(* Logix 5000 AddOnInstructionDefinition export Banner_Q5X_5000_Param_v4; software revision 33.00 *)

TYPE Banner_IOL_Port_v4 :   // UDT that has all of the data items necessary to communicate with a specific Port on a IO-Link Master
STRUCT
   Port_Controlled : INT;   // Each bit represents a port on an IO-Link Master. Set to 1 to tell AOI to control that port.
   Port_Activate : INT;   // Each bit represents a port on an IO-Link Master. When ON that port will process any commands in queue.
   Port_Read : INT;   // Each bit represents a port on an IO-Link Master. Used to determine when device AOI has requested a Read command.
   Port_Write : INT;   // Each bit represents a port on an IO-Link Master. Used to determine when device AOI has requested a Write command.
   Port_RW_Complete : INT;   // Each bit represents a port on an IO-Link Master. Tells device AOI that Read or Write request has been completed.
   Port_Device_Read : INT;
   Data_Transfer : SINT[190];   // Array to transfer data from IO-Master to device AOIs.
END_STRUCT
END_TYPE

TYPE Banner_Q5X_5000_RD_v4 :   // UDT that stores the Write Data for a Q5X 5000.
STRUCT
   Master_Cycle_Time : INT;
   Min_Cycle_Time : INT;
   M_Sequence_Capability : INT;
   IO_Link_Version_ID : INT;
   Process_Data_Input_Length : INT;
   Process_Data_Output_Length : INT;
   Combined_Vendor_ID : DINT;   // IO-Link Vendor ID
   Vendor_ID1 : INT;
   Vendor_ID2 : INT;
   Combined_Device_ID : DINT;   // IO-Link Device ID
   Device_ID1 : INT;
   Device_ID2 : INT;
   Device_ID3 : INT;
   Serial_Number : STRING;
   Teach_State : SINT;
   SP1_TP1 : SINT;
   SP1_TP2 : SINT;
   Measurement_1 : DINT;
   Excess_Gain : DINT;   // Amount of singla measured over the minimum threshold.
   Stability : SINT;
   Emitter_Status : SINT;   // 0 = Active, 1 = Inactive
   Laser_Fault_Status : SINT;   // 0 = No Fault, 1 = Fault Present
   BDC1_Totalizer_Counts : DINT;
   BDC2_Totalizer_Counts : DINT;
   Temperature : DINT;
   Last_Taught_Temperature : DINT;   // Internal Temperature the last time device was taught.
   All_Time_Run_Time : DINT;   // Read only counter that tracks the total time sensor has been running since manufacture. Value in Hours.
   Display : STRING;   // Last Display information
   MDC_Lower_Limit : DINT;
   MDC_Upper_Limit : DINT;
   MDC_Unit : INT;
   MDC_Scale : SINT;
END_STRUCT
END_TYPE

TYPE Banner_Q5X_5000_v4 :   // All of the parameters for a Q5X 5000.
STRUCT
   Initial_Global_Read : BOOL;   // Determines if all of the IO-Link data has been read into the PLC yet
   Command : INT;   // Value placed in here will activate a read or write to a specifc IO-Link Index
   Read : Banner_Q5X_5000_RD_v4;   // Read Only Data
   Write : Banner_Q5X_5000_WD_v4;   // Write Data
   Archive : Banner_Q5X_5000_WD_v4;   // Archive Data
   Reset : BOOL;   // Resets AOI. This will force a complete parameter read of the sensor.
END_STRUCT
END_TYPE

TYPE Banner_Q5X_5000_WD_v4 :   // UDT that stores the Write Data for a Q5X 5000.
STRUCT
   System_Command : INT;   // See IODD file for list of commands that can be activated via the System Command interface
   Parameter_Access_Lock : SINT;   // Write access to all parameters is prohibited while value is 1. Only this parameter can be adjusted when value is 1.
   Data_Storage_Lock : SINT;   // Automatic data storage is disabled when this value is equal to 1. Read access is not affected.
   Local_Parameterization_Lock : SINT;   // Parameterization via local control elements on device is disabled.
   Local_User_Interface_Lock : SINT;   // Operation of local user interface is disabled.
   Teach_in_Channel : SINT;   // 0 = Default, 1 = BDC1, 2 = BDC2
   BDC1_Setpoint_1 : DINT;
   BDC1_Setpoint_2 : DINT;   // In FGS, defines the second switching point. Other modes do not use this parameter.
   BDC1_Switchpoint_Logic : INT;   // 0 = Light Operate, 1 = Dark Operate
   BDC1_Mode : INT;   // 1 = 1Pt BGS, 128 = 2Pt Static BGS, 129 = Dynamic BGS, 130 = 1Pt Window (FGS), 131 = Dual Teach
   BDC1_Hysteresis : INT;   // Hysteresis value for the switchpoint. A value of 0 will result in automatically calculated hysteresis
   BDC2_Setpoint_1 : DINT;
   BDC2_Setpoint_2 : DINT;   // In FGS, defines the second switching point. Other modes do not use this parameter.
   BDC2_Switchpoint_Logic : INT;   // 0 = Light Operate, 1 = Dark Operate
   BDC2_Mode : INT;   // BDC1_Mode SINT Decimal 1 = 1Pt BGS, 128 = 2Pt Static BGS, 129 = Dynamic BGS, 130 = 1Pt Window (FGS), 131 = Dual Teach
   BDC2_Hysteresis : INT;   // Hysteresis value for the switchpoint. A value of 0 will result in automatically calculated hysteresis
   Response_Speed : SINT;   // 0 = Speed 0, 1 = Speed 1, 2 = Speed 2, 3 = Speed 3
   Gain : SINT;   // 0 = Normal, 1 = Best Accuracy, 2 = High Excess Gain
   Secondary_Output_Mode : SINT;   // 0 = Independent Output, 1 = Complementary Output, 2 = Pulse Frequency Output
   Zero_Reference_Location : SINT;   // 0 = Near, 1 = Far
   Shift_Zero_after_Teach : SINT;   // 0 = Off, 1 = On
   Display_Read : SINT;   // 0 = On, 1 = On Inverted, 2 = Off, 3 = Off Inverted
   Display_Units : SINT;   // 0 = Centimeters, 1 = Inches, 2 = Millimeters
   Pushbutton_Lockout : SINT;   // 0 = No Lockout, 1 = Pushbuttons Locked, 2 = Operator Lockout
   Output_Polarity : SINT;   // 0 = Default, 1 = PNP, 2 = NPN
   IOL_Filter_Time : INT;   // Time to average IOl process data measurement between updates
   Include_Binary : SINT;   // 0 = Include, 1 = Don't Include, 2= Measurement Device
   Measurement_1 : SINT;   // 0 = Disabled, 1 = Excess Gain, 2 = Excess Gain / 10, 3 = Channel 1 Dual Mode Percent
   Measurement_2 : SINT;   // 0 = Disabled, 1 = Distance Value, 2 = Displayed Distance, 3 = Channel 2 Dual Mode Percent
   BDC1_Delay_Mode : SINT;   // 0 = Disabled, 1 = On Off Delay, 2 = Oneshot, 3 = Totalizer
   BDC1_Delay_Timer_1 : DINT;   // 0 to 90000
   BDC1_Delay_Timer_2 : DINT;   // 0 to 90000
   BDC1_BGS_Teach_Offset : SINT;   // 0 = Auto, 1 = User Selected
   BDC1_FGS_Window_Size : SINT;   // 0 = Auto, 1 = User Selected
   BDC1_User_Teach_Offset : DINT;   // Mode must be FGS of BGS. Set the user defined offset. Can be positive or negative.
   BDC1_User_FGS_Window_Size : DINT;   // Mode must be FGS. Set the +/- window value.
   BDC1_Auto_Thresholding : SINT;   // 0 = On, 1 = Off, 2 = High Speed
   BDC2_Delay_Mode : SINT;   // 0 = Disabled, 1 = On Off Delay, 2 = Oneshot, 3 = Totalizer
   BDC2_Delay_Timer_1 : DINT;   // 0 to 90000
   BDC2_Delay_Timer_2 : DINT;   // 0 to 90000
   BDC2_BGS_Teach_Offset : SINT;   // 0 = Auto, 1 = User Selected
   BDC2_FGS_Window_Size : SINT;   // 0 = Auto, 1 = User Selected
   BDC2_User_Teach_Offset : DINT;   // Mode must be FGS of BGS. Set the user defined offset. Can be positive or negative.
   BDC2_User_FGS_Window_Size : DINT;   // Mode must be FGS. Set the +/- window value.
   BDC2_Auto_Thresholding : SINT;   // 0 = On, 1 = Off, 2 = High Speed
   Resettable_Run_Time : DINT;
   PFM_Near : DINT;   // 100 to 45000 in Hz
   PFM_Far : DINT;   // 100 to 45000 in Hz
   All_Time_Run_Time_Event_Time : DINT;
   Resettable_Run_Time_Event_Time : DINT;
END_STRUCT
END_TYPE

ADD_ON_INSTRUCTION Banner_Q5X_5000_Param_v4   (* revision 4.1, vendor Banner Engineering *)
// AOI to read and write parameter data to an IO-Link Q5X.
VAR_IN_OUT
   Q5X : Banner_Q5X_5000_v4; {required}
   Port_Data : Banner_IOL_Port_v4; {required}
END_VAR
VAR_INPUT
   Port : DINT; {required}
END_VAR
VAR
   Local_Control : DINT; {access None}
   Global_Read_Command_Value : INT; {access None}
   Global_Write_Command_Value : INT; {access None}
   Command_Being_Processed : BOOL; {access None}
   Update_Archive : BOOL; {access None}
   Index_Write_Inprocess : INT; {access None}
   Index_Write_Control : INT; {access None}
   Inprocess_Index : DINT; {access None}
END_VAR

ROUTINE Logic   (* ladder *)
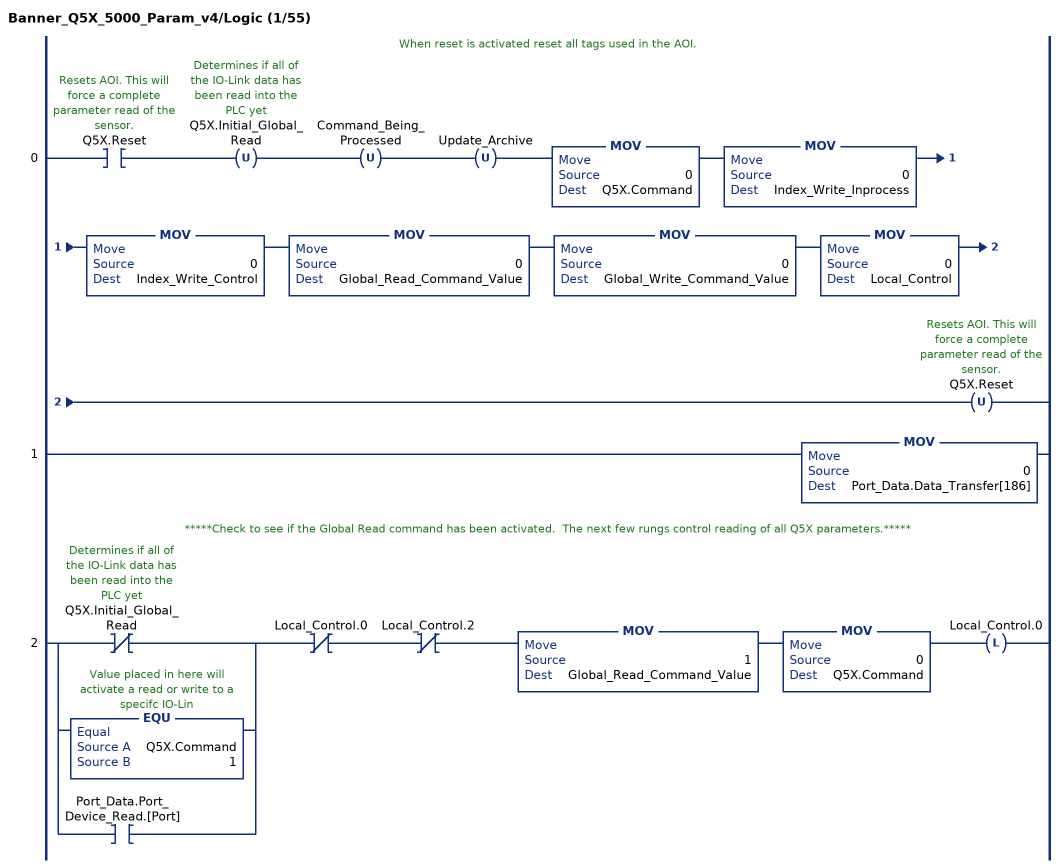
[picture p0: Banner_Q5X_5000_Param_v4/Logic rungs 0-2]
   // When reset is activated reset all tags used in the AOI.
   0: XIC(Q5X.Reset)OTU(Q5X.Initial_Global_Read)OTU(Command_Being_Processed)OTU(Update_Archive)MOV(0,Q5X.Command)MOV(0,Index_Write_Inprocess)MOV(0,Index_Write_Control)MOV(0,Global_Read_Command_Value)MOV(0,Global_Write_Command_Value)MOV(0,Local_Control)OTU(Q5X.Reset);
   1: MOV(0,Port_Data.Data_Transfer[186]);
   // *****Check to see if the Global Read command has been activated.  The next few rungs control reading of all Q5X parameters.*****
   2: [XIO(Q5X.Initial_Global_Read) ,EQU(Q5X.Command,1) ,XIC(Port_Data.Port_Device_Read.[Port]) ]XIO(Local_Control.0)XIO(Local_Control.2)MOV(1,Global_Read_Command_Value)MOV(0,Q5X.Command)OTL(Local_Control.0);
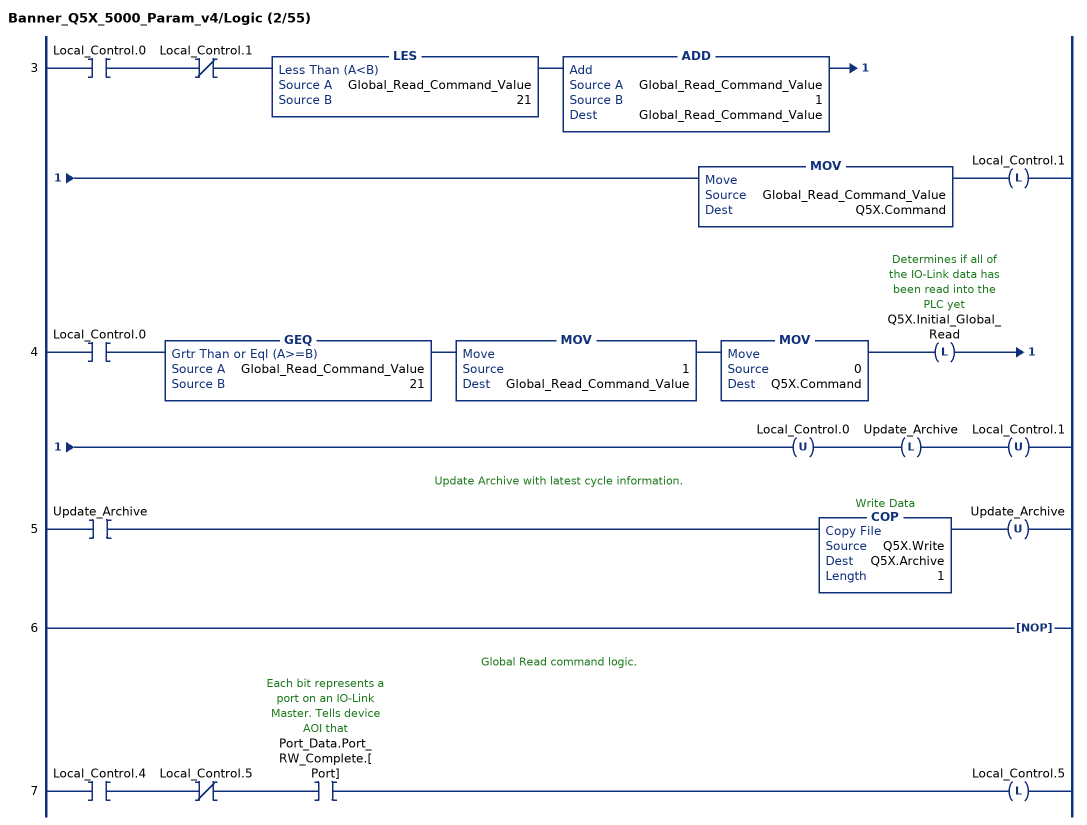
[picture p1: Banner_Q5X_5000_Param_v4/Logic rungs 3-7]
   3: XIC(Local_Control.0)XIO(Local_Control.1)LES(Global_Read_Command_Value,21)ADD(Global_Read_Command_Value,1,Global_Read_Command_Value)MOV(Global_Read_Command_Value,Q5X.Command)OTL(Local_Control.1);
   4: XIC(Local_Control.0)GEQ(Global_Read_Command_Value,21)MOV(1,Global_Read_Command_Value)MOV(0,Q5X.Command)OTL(Q5X.Initial_Global_Read)OTU(Local_Control.0)OTL(Update_Archive)OTU(Local_Control.1);
   // Update Archive with latest cycle information.
   5: XIC(Update_Archive)COP(Q5X.Write,Q5X.Archive,1)OTU(Update_Archive);
   6: NOP();
   // Global Read command logic.
   7: XIC(Local_Control.4)XIO(Local_Control.5)XIC(Port_Data.Port_RW_Complete.[Port])OTL(Local_Control.5);
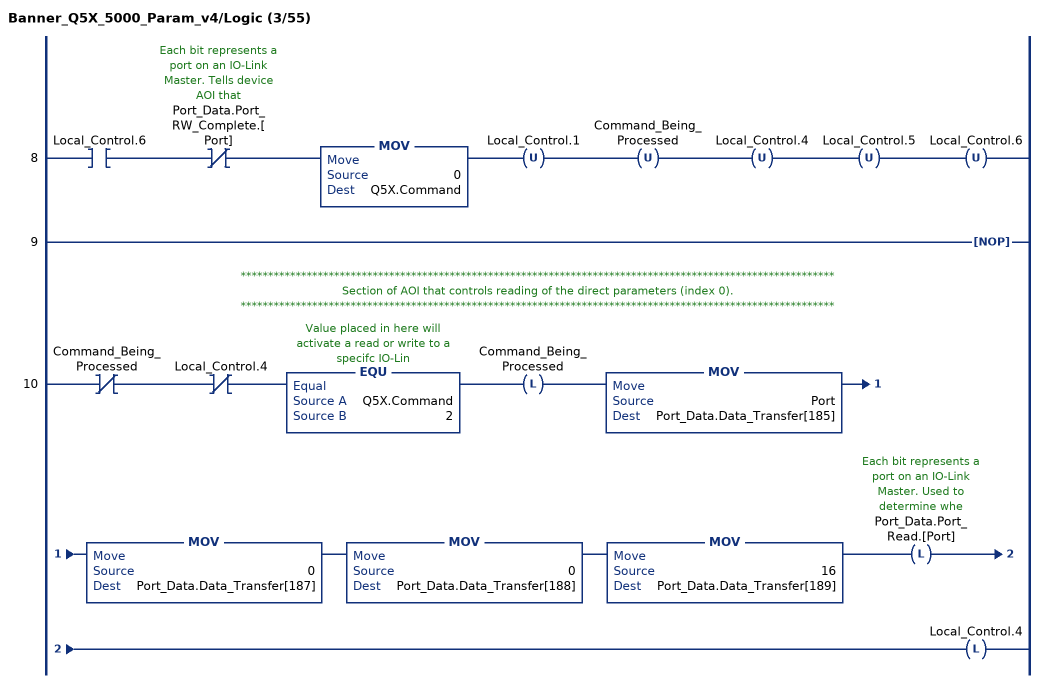
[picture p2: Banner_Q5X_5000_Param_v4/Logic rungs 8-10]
   8: XIC(Local_Control.6)XIO(Port_Data.Port_RW_Complete.[Port])MOV(0,Q5X.Command)OTU(Local_Control.1)OTU(Command_Being_Processed)OTU(Local_Control.4)OTU(Local_Control.5)OTU(Local_Control.6);
   9: NOP();
   // ************************************************************************************************************
   // Section of AOI that controls reading of the direct parameters (index 0).
   // ************************************************************************************************************
   10: XIO(Command_Being_Processed)XIO(Local_Control.4)EQU(Q5X.Command,2)OTL(Command_Being_Processed)MOV(Port,Port_Data.Data_Transfer[185])MOV(0,Port_Data.Data_Transfer[187])MOV(0,Port_Data.Data_Transfer[188])MOV(16,Port_Data.Data_Transfer[189])OTL(Port_Data.Port_Read.[Port])OTL(Local_Control.4);
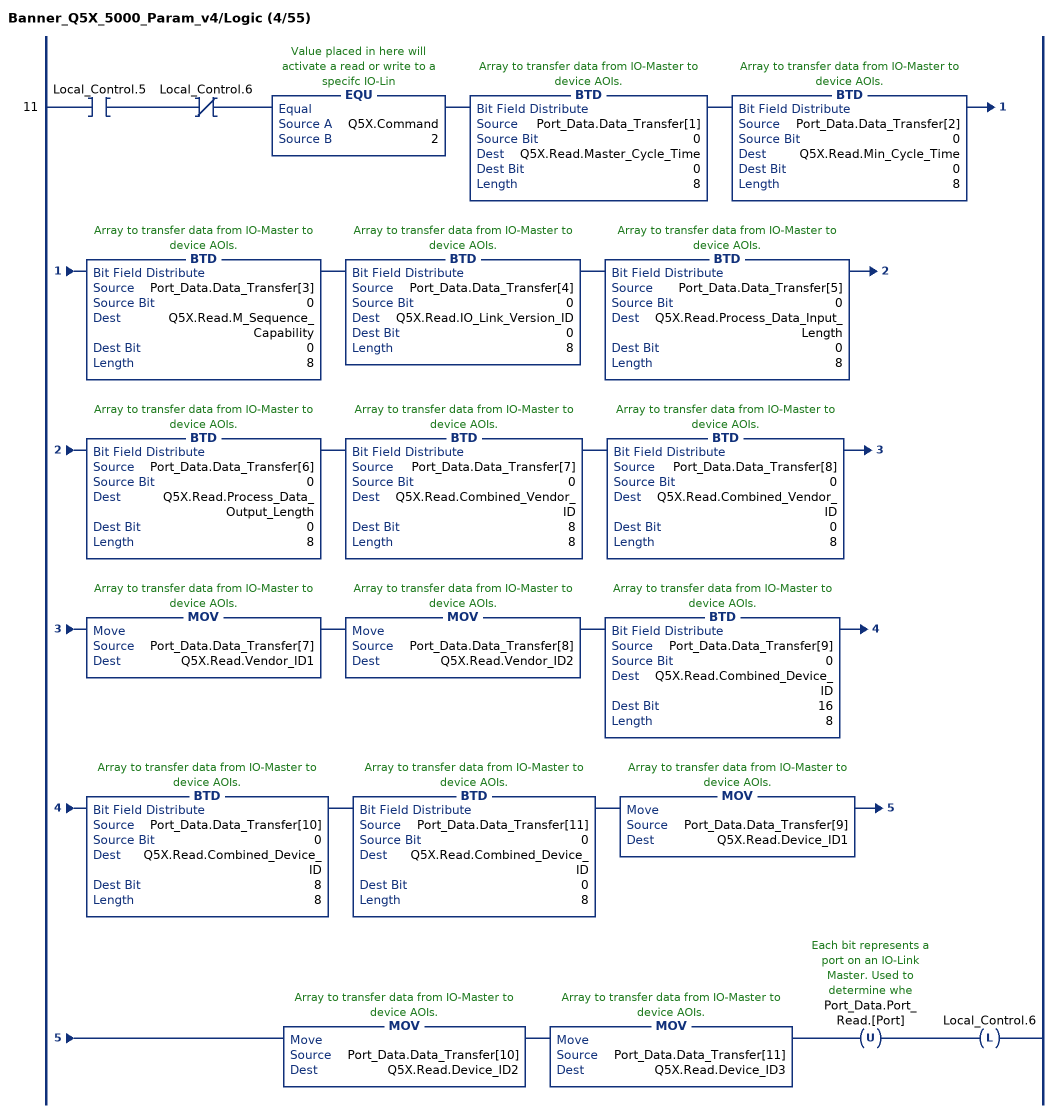
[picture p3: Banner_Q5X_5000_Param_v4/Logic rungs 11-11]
   11: XIC(Local_Control.5)XIO(Local_Control.6)EQU(Q5X.Command,2)BTD(Port_Data.Data_Transfer[1],0,Q5X.Read.Master_Cycle_Time,0,8)BTD(Port_Data.Data_Transfer[2],0,Q5X.Read.Min_Cycle_Time,0,8)BTD(Port_Data.Data_Transfer[3],0,Q5X.Read.M_Sequence_Capability,0,8)BTD(Port_Data.Data_Transfer[4],0,Q5X.Read.IO_Link_Version_ID,0,8)BTD(Port_Data.Data_Transfer[5],0,Q5X.Read.Process_Data_Input_Length,0,8)BTD(Port_Data.Data_Transfer[6],0,Q5X.Read.Process_Data_Output_Length,0,8)BTD(Port_Data.Data_Transfer[7],0,Q5X.Read.Combined_Vendor_ID,8,8)BTD(Port_Data.Data_Transfer[8],0,Q5X.Read.Combined_Vendor_ID,0,8)MOV(Port_Data.Data_Transfer[7],Q5X.Read.Vendor_ID1)MOV(Port_Data.Data_Transfer[8],Q5X.Read.Vendor_ID2)BTD(Port_Data.Data_Transfer[9],0,Q5X.Read.Combined_Device_ID,16,8)BTD(Port_Data.Data_Transfer[10],0,Q5X.Read.Combined_Device_ID,8,8)BTD(Port_Data.Data_Transfer[11],0,Q5X.Read.Combined_Device_ID,0,8)MOV(Port_Data.Data_Transfer[9],Q5X.Read.Device_ID1)MOV(Port_Data.Data_Transfer[10],Q5X.Read.Device_ID2)MOV(Port_Data.Data_Transfer[11],Q5X.Read.Device_ID3)OTU(Port_Data.Port_Read.[Port])OTL(Local_Control.6);
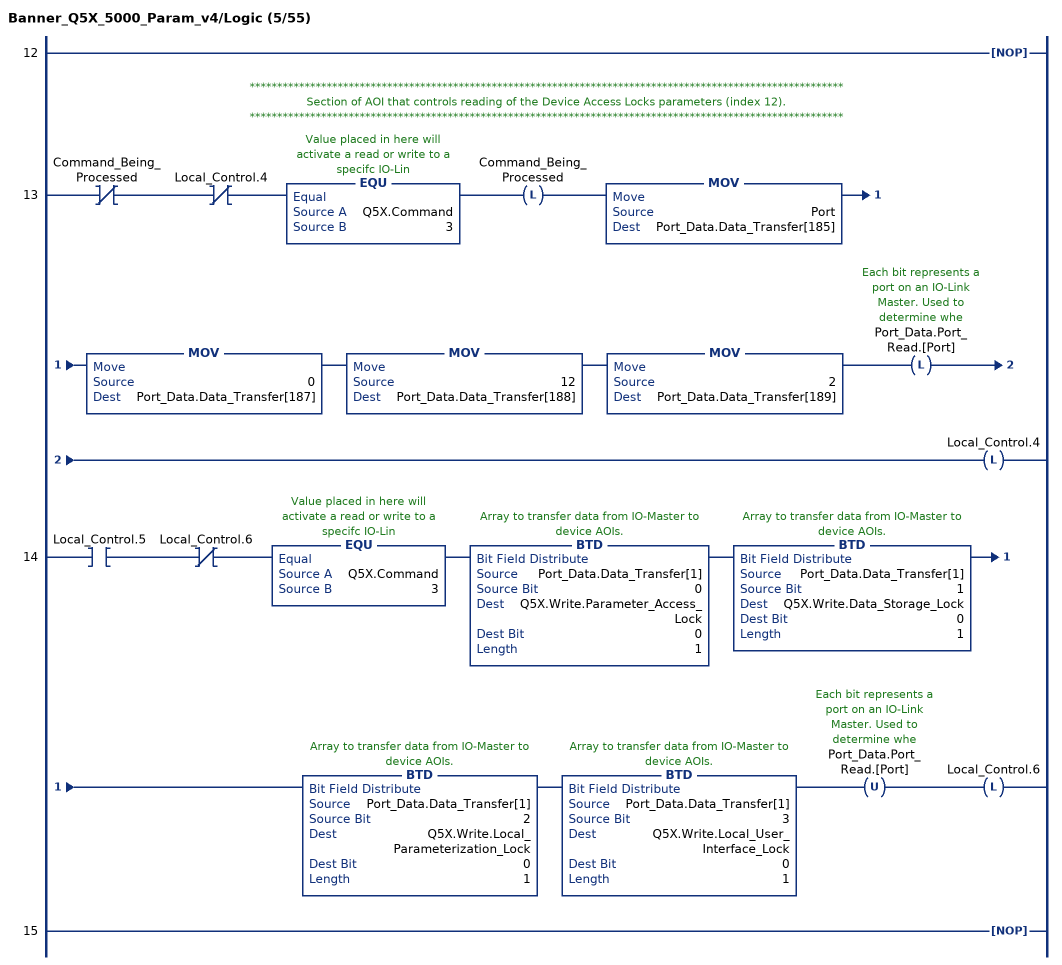
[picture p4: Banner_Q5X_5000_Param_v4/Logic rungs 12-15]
   12: NOP();
   // ************************************************************************************************************
   // Section of AOI that controls reading of the Device Access Locks parameters (index 12).
   // ************************************************************************************************************
   13: XIO(Command_Being_Processed)XIO(Local_Control.4)EQU(Q5X.Command,3)OTL(Command_Being_Processed)MOV(Port,Port_Data.Data_Transfer[185])MOV(0,Port_Data.Data_Transfer[187])MOV(12,Port_Data.Data_Transfer[188])MOV(2,Port_Data.Data_Transfer[189])OTL(Port_Data.Port_Read.[Port])OTL(Local_Control.4);
   14: XIC(Local_Control.5)XIO(Local_Control.6)EQU(Q5X.Command,3)BTD(Port_Data.Data_Transfer[1],0,Q5X.Write.Parameter_Access_Lock,0,1)BTD(Port_Data.Data_Transfer[1],1,Q5X.Write.Data_Storage_Lock,0,1)BTD(Port_Data.Data_Transfer[1],2,Q5X.Write.Local_Parameterization_Lock,0,1)BTD(Port_Data.Data_Transfer[1],3,Q5X.Write.Local_User_Interface_Lock,0,1)OTU(Port_Data.Port_Read.[Port])OTL(Local_Control.6);
   15: NOP();
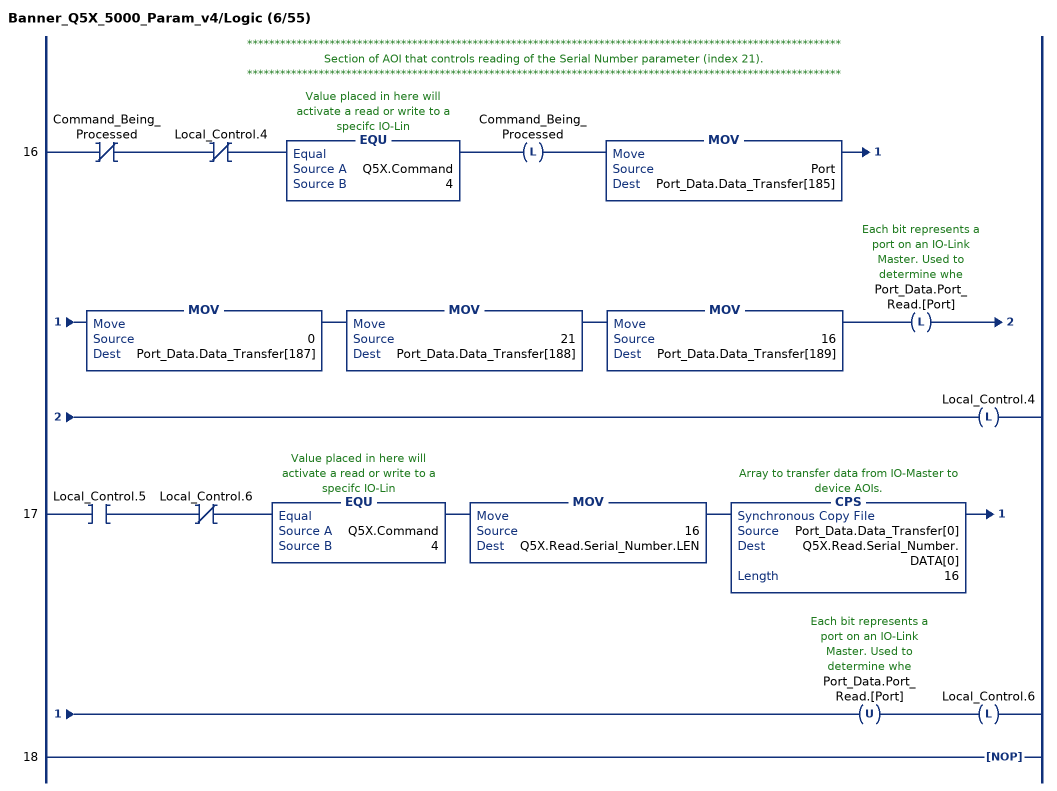
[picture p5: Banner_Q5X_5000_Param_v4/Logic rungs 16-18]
   // ************************************************************************************************************
   // Section of AOI that controls reading of the Serial Number parameter (index 21).
   // ************************************************************************************************************
   16: XIO(Command_Being_Processed)XIO(Local_Control.4)EQU(Q5X.Command,4)OTL(Command_Being_Processed)MOV(Port,Port_Data.Data_Transfer[185])MOV(0,Port_Data.Data_Transfer[187])MOV(21,Port_Data.Data_Transfer[188])MOV(16,Port_Data.Data_Transfer[189])OTL(Port_Data.Port_Read.[Port])OTL(Local_Control.4);
   17: XIC(Local_Control.5)XIO(Local_Control.6)EQU(Q5X.Command,4)MOV(16,Q5X.Read.Serial_Number.LEN)CPS(Port_Data.Data_Transfer[0],Q5X.Read.Serial_Number.DATA[0],16)OTU(Port_Data.Port_Read.[Port])OTL(Local_Control.6);
   18: NOP();
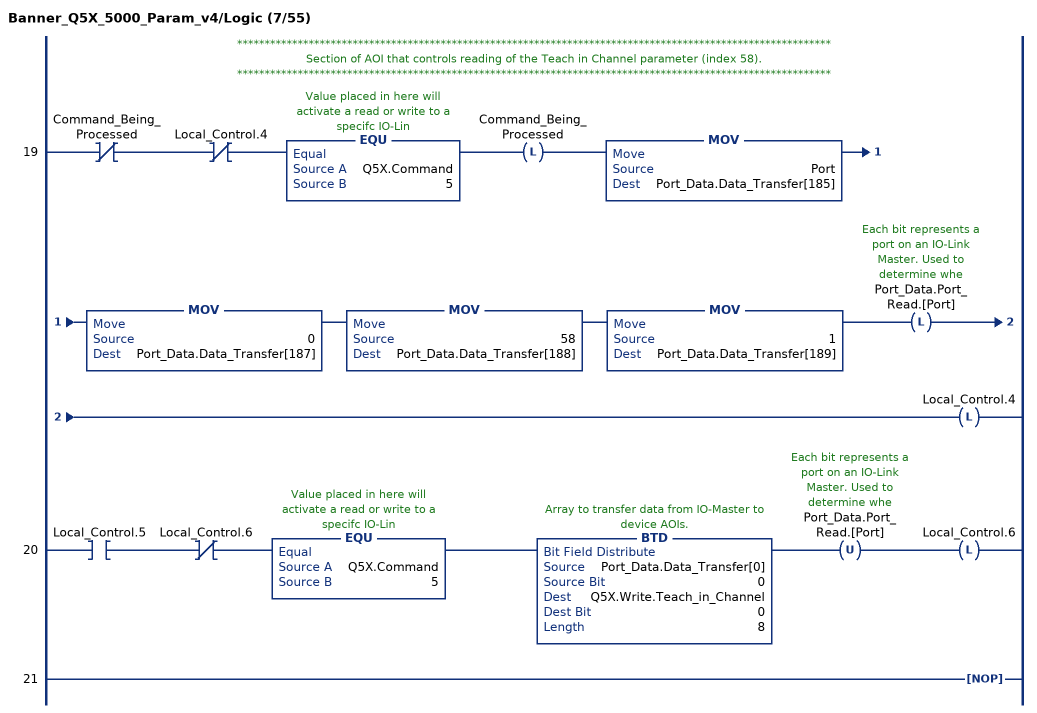
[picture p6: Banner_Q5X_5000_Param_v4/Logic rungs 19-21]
   // ************************************************************************************************************
   // Section of AOI that controls reading of the Teach in Channel parameter (index 58).
   // ************************************************************************************************************
   19: XIO(Command_Being_Processed)XIO(Local_Control.4)EQU(Q5X.Command,5)OTL(Command_Being_Processed)MOV(Port,Port_Data.Data_Transfer[185])MOV(0,Port_Data.Data_Transfer[187])MOV(58,Port_Data.Data_Transfer[188])MOV(1,Port_Data.Data_Transfer[189])OTL(Port_Data.Port_Read.[Port])OTL(Local_Control.4);
   20: XIC(Local_Control.5)XIO(Local_Control.6)EQU(Q5X.Command,5)BTD(Port_Data.Data_Transfer[0],0,Q5X.Write.Teach_in_Channel,0,8)OTU(Port_Data.Port_Read.[Port])OTL(Local_Control.6);
   21: NOP();
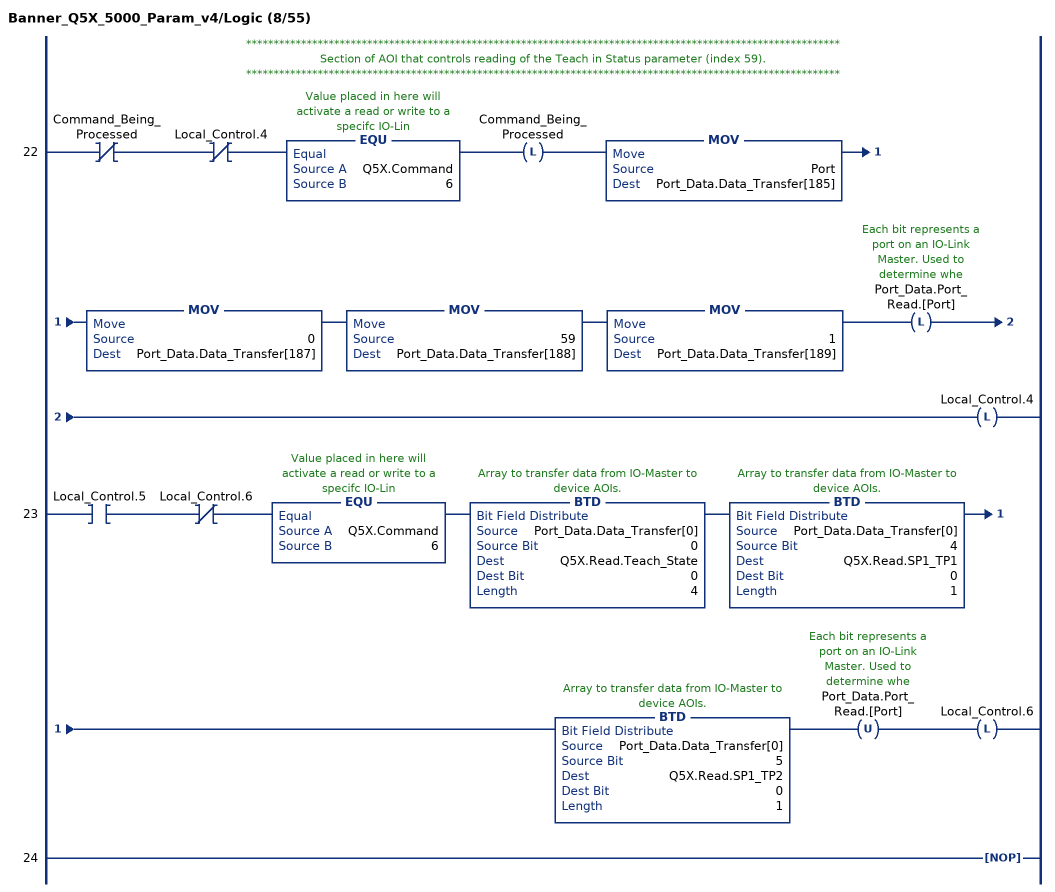
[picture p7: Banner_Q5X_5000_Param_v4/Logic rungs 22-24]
   // ************************************************************************************************************
   // Section of AOI that controls reading of the Teach in Status parameter (index 59).
   // ************************************************************************************************************
   22: XIO(Command_Being_Processed)XIO(Local_Control.4)EQU(Q5X.Command,6)OTL(Command_Being_Processed)MOV(Port,Port_Data.Data_Transfer[185])MOV(0,Port_Data.Data_Transfer[187])MOV(59,Port_Data.Data_Transfer[188])MOV(1,Port_Data.Data_Transfer[189])OTL(Port_Data.Port_Read.[Port])OTL(Local_Control.4);
   23: XIC(Local_Control.5)XIO(Local_Control.6)EQU(Q5X.Command,6)BTD(Port_Data.Data_Transfer[0],0,Q5X.Read.Teach_State,0,4)BTD(Port_Data.Data_Transfer[0],4,Q5X.Read.SP1_TP1,0,1)BTD(Port_Data.Data_Transfer[0],5,Q5X.Read.SP1_TP2,0,1)OTU(Port_Data.Port_Read.[Port])OTL(Local_Control.6);
   24: NOP();
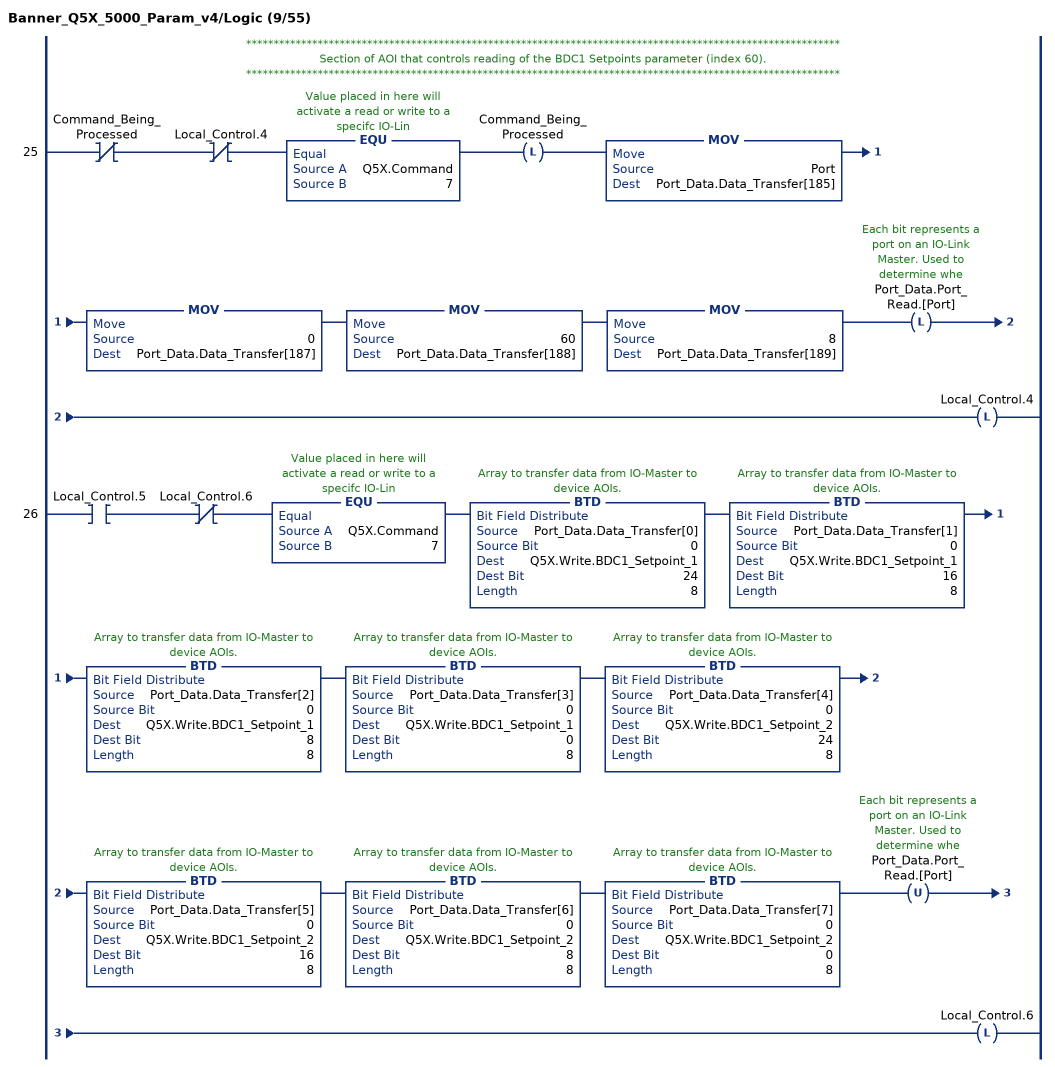
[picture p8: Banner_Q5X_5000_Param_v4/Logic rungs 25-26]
   // ************************************************************************************************************
   // Section of AOI that controls reading of the BDC1 Setpoints parameter (index 60).
   // ************************************************************************************************************
   25: XIO(Command_Being_Processed)XIO(Local_Control.4)EQU(Q5X.Command,7)OTL(Command_Being_Processed)MOV(Port,Port_Data.Data_Transfer[185])MOV(0,Port_Data.Data_Transfer[187])MOV(60,Port_Data.Data_Transfer[188])MOV(8,Port_Data.Data_Transfer[189])OTL(Port_Data.Port_Read.[Port])OTL(Local_Control.4);
   26: XIC(Local_Control.5)XIO(Local_Control.6)EQU(Q5X.Command,7)BTD(Port_Data.Data_Transfer[0],0,Q5X.Write.BDC1_Setpoint_1,24,8)BTD(Port_Data.Data_Transfer[1],0,Q5X.Write.BDC1_Setpoint_1,16,8)BTD(Port_Data.Data_Transfer[2],0,Q5X.Write.BDC1_Setpoint_1,8,8)BTD(Port_Data.Data_Transfer[3],0,Q5X.Write.BDC1_Setpoint_1,0,8)BTD(Port_Data.Data_Transfer[4],0,Q5X.Write.BDC1_Setpoint_2,24,8)BTD(Port_Data.Data_Transfer[5],0,Q5X.Write.BDC1_Setpoint_2,16,8)BTD(Port_Data.Data_Transfer[6],0,Q5X.Write.BDC1_Setpoint_2,8,8)BTD(Port_Data.Data_Transfer[7],0,Q5X.Write.BDC1_Setpoint_2,0,8)OTU(Port_Data.Port_Read.[Port])OTL(Local_Control.6);
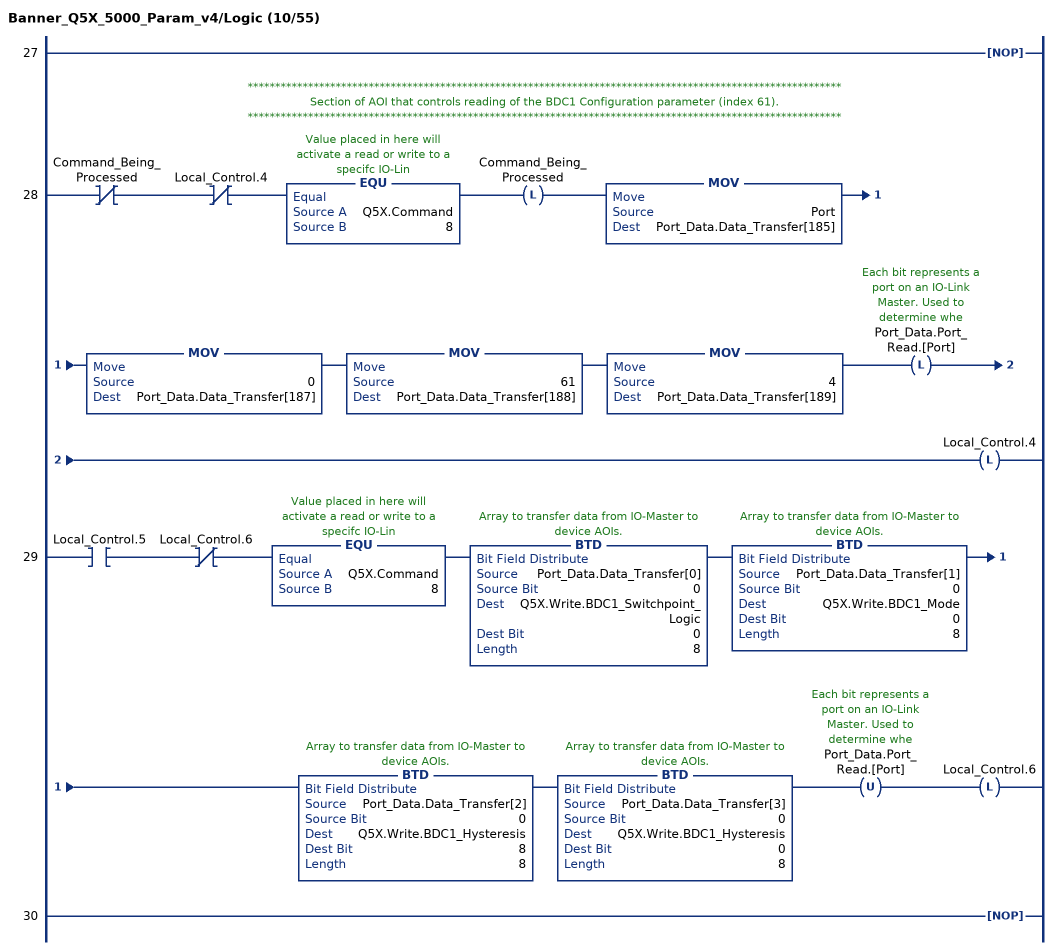
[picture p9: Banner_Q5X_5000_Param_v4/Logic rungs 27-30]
   27: NOP();
   // ************************************************************************************************************
   // Section of AOI that controls reading of the BDC1 Configuration parameter (index 61).
   // ************************************************************************************************************
   28: XIO(Command_Being_Processed)XIO(Local_Control.4)EQU(Q5X.Command,8)OTL(Command_Being_Processed)MOV(Port,Port_Data.Data_Transfer[185])MOV(0,Port_Data.Data_Transfer[187])MOV(61,Port_Data.Data_Transfer[188])MOV(4,Port_Data.Data_Transfer[189])OTL(Port_Data.Port_Read.[Port])OTL(Local_Control.4);
   29: XIC(Local_Control.5)XIO(Local_Control.6)EQU(Q5X.Command,8)BTD(Port_Data.Data_Transfer[0],0,Q5X.Write.BDC1_Switchpoint_Logic,0,8)BTD(Port_Data.Data_Transfer[1],0,Q5X.Write.BDC1_Mode,0,8)BTD(Port_Data.Data_Transfer[2],0,Q5X.Write.BDC1_Hysteresis,8,8)BTD(Port_Data.Data_Transfer[3],0,Q5X.Write.BDC1_Hysteresis,0,8)OTU(Port_Data.Port_Read.[Port])OTL(Local_Control.6);
   30: NOP();
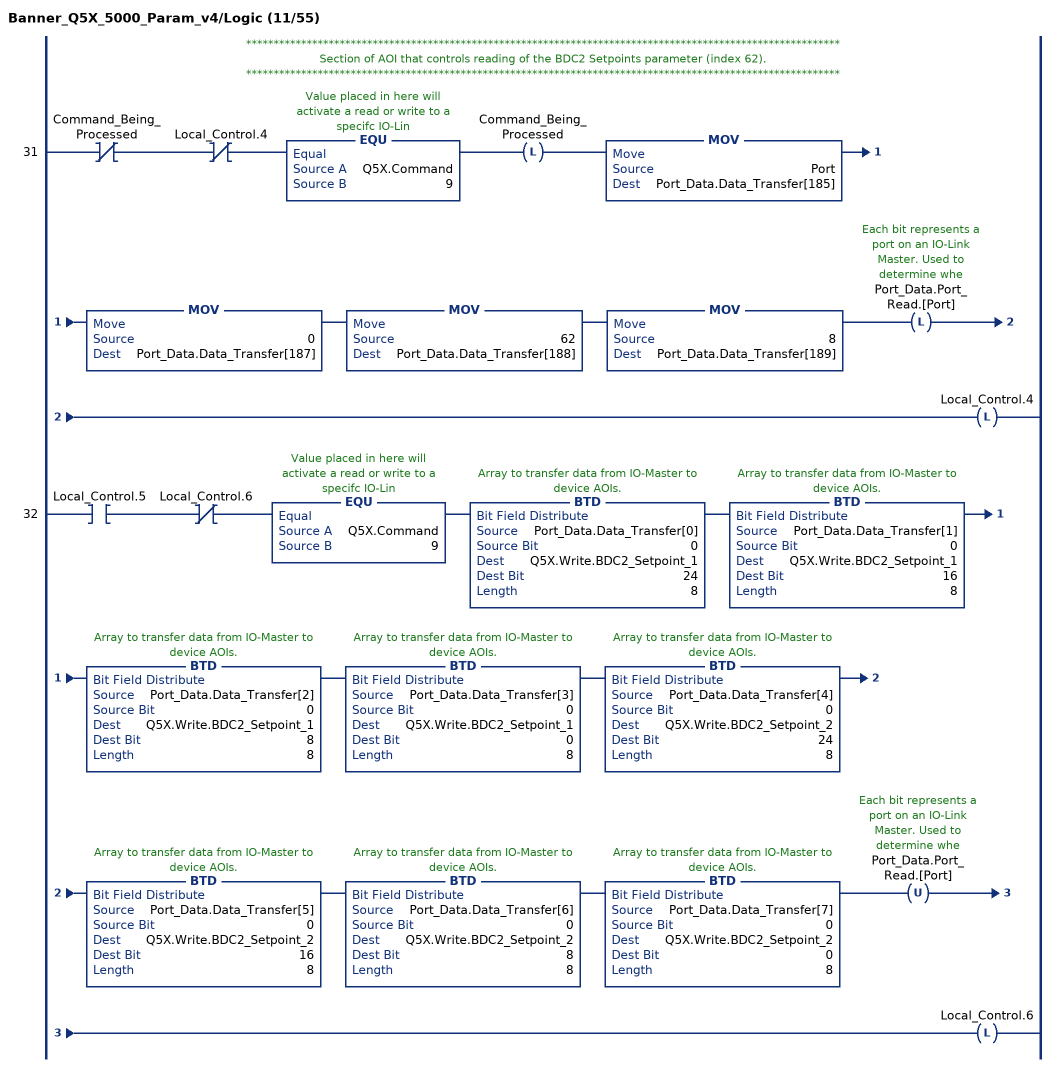
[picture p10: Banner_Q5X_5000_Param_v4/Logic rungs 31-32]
   // ************************************************************************************************************
   // Section of AOI that controls reading of the BDC2 Setpoints parameter (index 62).
   // ************************************************************************************************************
   31: XIO(Command_Being_Processed)XIO(Local_Control.4)EQU(Q5X.Command,9)OTL(Command_Being_Processed)MOV(Port,Port_Data.Data_Transfer[185])MOV(0,Port_Data.Data_Transfer[187])MOV(62,Port_Data.Data_Transfer[188])MOV(8,Port_Data.Data_Transfer[189])OTL(Port_Data.Port_Read.[Port])OTL(Local_Control.4);
   32: XIC(Local_Control.5)XIO(Local_Control.6)EQU(Q5X.Command,9)BTD(Port_Data.Data_Transfer[0],0,Q5X.Write.BDC2_Setpoint_1,24,8)BTD(Port_Data.Data_Transfer[1],0,Q5X.Write.BDC2_Setpoint_1,16,8)BTD(Port_Data.Data_Transfer[2],0,Q5X.Write.BDC2_Setpoint_1,8,8)BTD(Port_Data.Data_Transfer[3],0,Q5X.Write.BDC2_Setpoint_1,0,8)BTD(Port_Data.Data_Transfer[4],0,Q5X.Write.BDC2_Setpoint_2,24,8)BTD(Port_Data.Data_Transfer[5],0,Q5X.Write.BDC2_Setpoint_2,16,8)BTD(Port_Data.Data_Transfer[6],0,Q5X.Write.BDC2_Setpoint_2,8,8)BTD(Port_Data.Data_Transfer[7],0,Q5X.Write.BDC2_Setpoint_2,0,8)OTU(Port_Data.Port_Read.[Port])OTL(Local_Control.6);
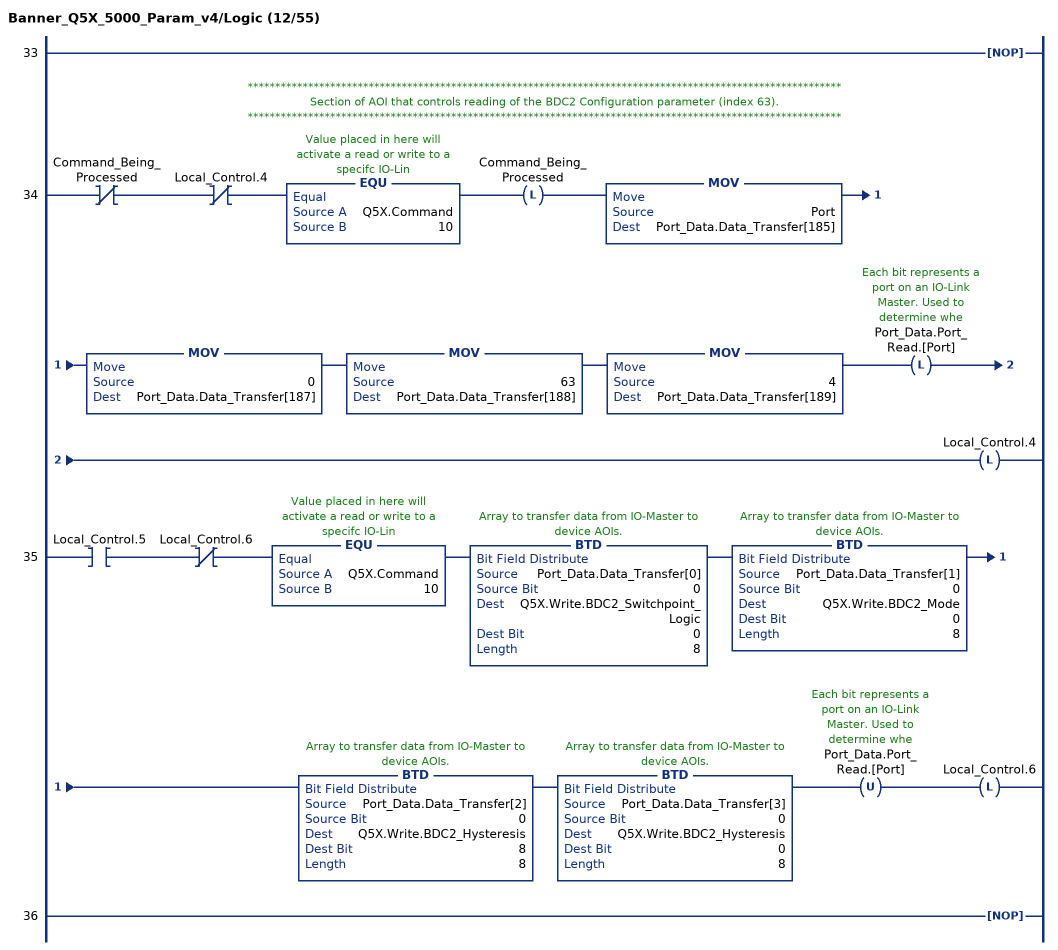
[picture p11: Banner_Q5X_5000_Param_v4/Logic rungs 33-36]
   33: NOP();
   // ************************************************************************************************************
   // Section of AOI that controls reading of the BDC2 Configuration parameter (index 63).
   // ************************************************************************************************************
   34: XIO(Command_Being_Processed)XIO(Local_Control.4)EQU(Q5X.Command,10)OTL(Command_Being_Processed)MOV(Port,Port_Data.Data_Transfer[185])MOV(0,Port_Data.Data_Transfer[187])MOV(63,Port_Data.Data_Transfer[188])MOV(4,Port_Data.Data_Transfer[189])OTL(Port_Data.Port_Read.[Port])OTL(Local_Control.4);
   35: XIC(Local_Control.5)XIO(Local_Control.6)EQU(Q5X.Command,10)BTD(Port_Data.Data_Transfer[0],0,Q5X.Write.BDC2_Switchpoint_Logic,0,8)BTD(Port_Data.Data_Transfer[1],0,Q5X.Write.BDC2_Mode,0,8)BTD(Port_Data.Data_Transfer[2],0,Q5X.Write.BDC2_Hysteresis,8,8)BTD(Port_Data.Data_Transfer[3],0,Q5X.Write.BDC2_Hysteresis,0,8)OTU(Port_Data.Port_Read.[Port])OTL(Local_Control.6);
   36: NOP();
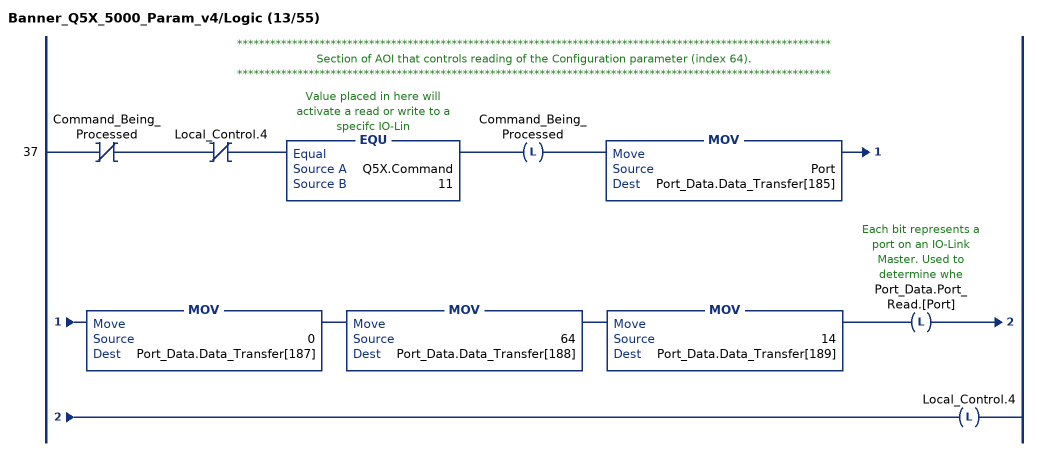
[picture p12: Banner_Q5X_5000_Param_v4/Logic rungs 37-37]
   // ************************************************************************************************************
   // Section of AOI that controls reading of the Configuration parameter (index 64).
   // ************************************************************************************************************
   37: XIO(Command_Being_Processed)XIO(Local_Control.4)EQU(Q5X.Command,11)OTL(Command_Being_Processed)MOV(Port,Port_Data.Data_Transfer[185])MOV(0,Port_Data.Data_Transfer[187])MOV(64,Port_Data.Data_Transfer[188])MOV(14,Port_Data.Data_Transfer[189])OTL(Port_Data.Port_Read.[Port])OTL(Local_Control.4);
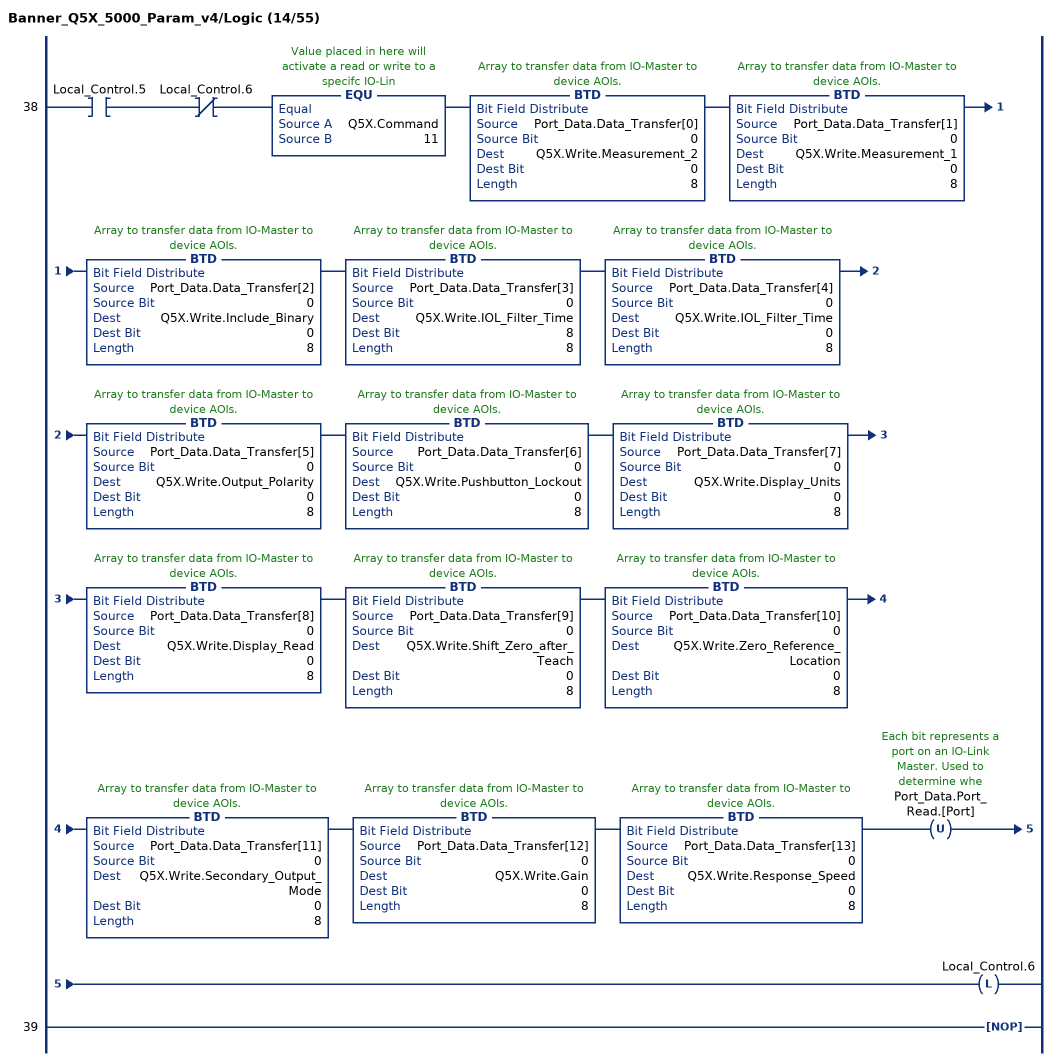
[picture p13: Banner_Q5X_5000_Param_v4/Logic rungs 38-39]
   38: XIC(Local_Control.5)XIO(Local_Control.6)EQU(Q5X.Command,11)BTD(Port_Data.Data_Transfer[0],0,Q5X.Write.Measurement_2,0,8)BTD(Port_Data.Data_Transfer[1],0,Q5X.Write.Measurement_1,0,8)BTD(Port_Data.Data_Transfer[2],0,Q5X.Write.Include_Binary,0,8)BTD(Port_Data.Data_Transfer[3],0,Q5X.Write.IOL_Filter_Time,8,8)BTD(Port_Data.Data_Transfer[4],0,Q5X.Write.IOL_Filter_Time,0,8)BTD(Port_Data.Data_Transfer[5],0,Q5X.Write.Output_Polarity,0,8)BTD(Port_Data.Data_Transfer[6],0,Q5X.Write.Pushbutton_Lockout,0,8)BTD(Port_Data.Data_Transfer[7],0,Q5X.Write.Display_Units,0,8)BTD(Port_Data.Data_Transfer[8],0,Q5X.Write.Display_Read,0,8)BTD(Port_Data.Data_Transfer[9],0,Q5X.Write.Shift_Zero_after_Teach,0,8)BTD(Port_Data.Data_Transfer[10],0,Q5X.Write.Zero_Reference_Location,0,8)BTD(Port_Data.Data_Transfer[11],0,Q5X.Write.Secondary_Output_Mode,0,8)BTD(Port_Data.Data_Transfer[12],0,Q5X.Write.Gain,0,8)BTD(Port_Data.Data_Transfer[13],0,Q5X.Write.Response_Speed,0,8)OTU(Port_Data.Port_Read.[Port])OTL(Local_Control.6);
   39: NOP();
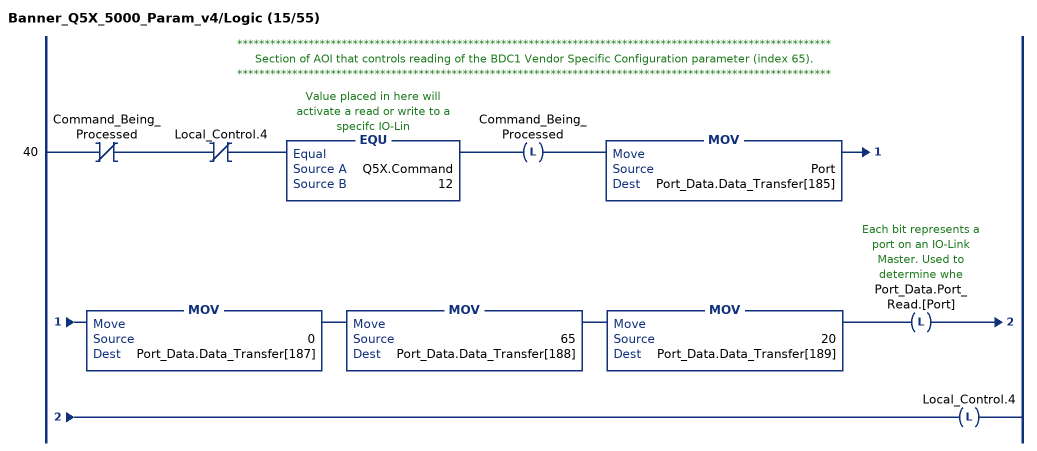
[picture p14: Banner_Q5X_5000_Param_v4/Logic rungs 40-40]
   // ************************************************************************************************************
   // Section of AOI that controls reading of the BDC1 Vendor Specific Configuration parameter (index 65).
   // ************************************************************************************************************
   40: XIO(Command_Being_Processed)XIO(Local_Control.4)EQU(Q5X.Command,12)OTL(Command_Being_Processed)MOV(Port,Port_Data.Data_Transfer[185])MOV(0,Port_Data.Data_Transfer[187])MOV(65,Port_Data.Data_Transfer[188])MOV(20,Port_Data.Data_Transfer[189])OTL(Port_Data.Port_Read.[Port])OTL(Local_Control.4);
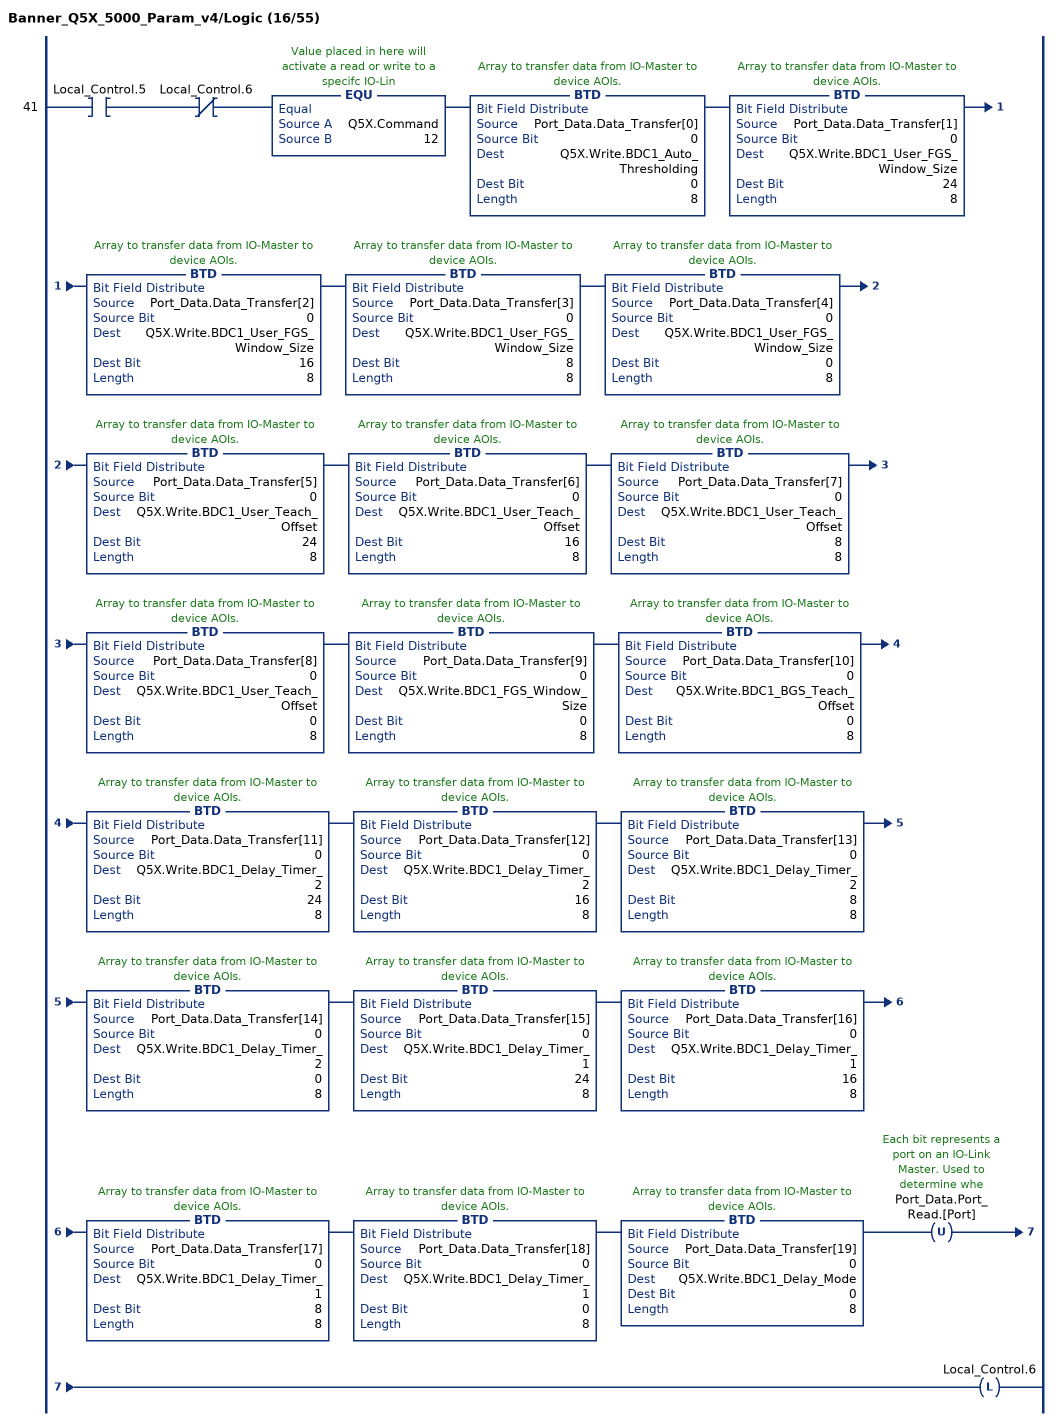
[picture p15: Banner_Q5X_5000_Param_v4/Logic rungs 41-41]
   41: XIC(Local_Control.5)XIO(Local_Control.6)EQU(Q5X.Command,12)BTD(Port_Data.Data_Transfer[0],0,Q5X.Write.BDC1_Auto_Thresholding,0,8)BTD(Port_Data.Data_Transfer[1],0,Q5X.Write.BDC1_User_FGS_Window_Size,24,8)BTD(Port_Data.Data_Transfer[2],0,Q5X.Write.BDC1_User_FGS_Window_Size,16,8)BTD(Port_Data.Data_Transfer[3],0,Q5X.Write.BDC1_User_FGS_Window_Size,8,8)BTD(Port_Data.Data_Transfer[4],0,Q5X.Write.BDC1_User_FGS_Window_Size,0,8)BTD(Port_Data.Data_Transfer[5],0,Q5X.Write.BDC1_User_Teach_Offset,24,8)BTD(Port_Data.Data_Transfer[6],0,Q5X.Write.BDC1_User_Teach_Offset,16,8)BTD(Port_Data.Data_Transfer[7],0,Q5X.Write.BDC1_User_Teach_Offset,8,8)BTD(Port_Data.Data_Transfer[8],0,Q5X.Write.BDC1_User_Teach_Offset,0,8)BTD(Port_Data.Data_Transfer[9],0,Q5X.Write.BDC1_FGS_Window_Size,0,8)BTD(Port_Data.Data_Transfer[10],0,Q5X.Write.BDC1_BGS_Teach_Offset,0,8)BTD(Port_Data.Data_Transfer[11],0,Q5X.Write.BDC1_Delay_Timer_2,24,8)BTD(Port_Data.Data_Transfer[12],0,Q5X.Write.BDC1_Delay_Timer_2,16,8)BTD(Port_Data.Data_Transfer[13],0,Q5X.Write.BDC1_Delay_Timer_2,8,8)BTD(Port_Data.Data_Transfer[14],0,Q5X.Write.BDC1_Delay_Timer_2,0,8)BTD(Port_Data.Data_Transfer[15],0,Q5X.Write.BDC1_Delay_Timer_1,24,8)BTD(Port_Data.Data_Transfer[16],0,Q5X.Write.BDC1_Delay_Timer_1,16,8)BTD(Port_Data.Data_Transfer[17],0,Q5X.Write.BDC1_Delay_Timer_1,8,8)BTD(Port_Data.Data_Transfer[18],0,Q5X.Write.BDC1_Delay_Timer_1,0,8)BTD(Port_Data.Data_Transfer[19],0,Q5X.Write.BDC1_Delay_Mode,0,8)OTU(Port_Data.Port_Read.[Port])OTL(Local_Control.6);
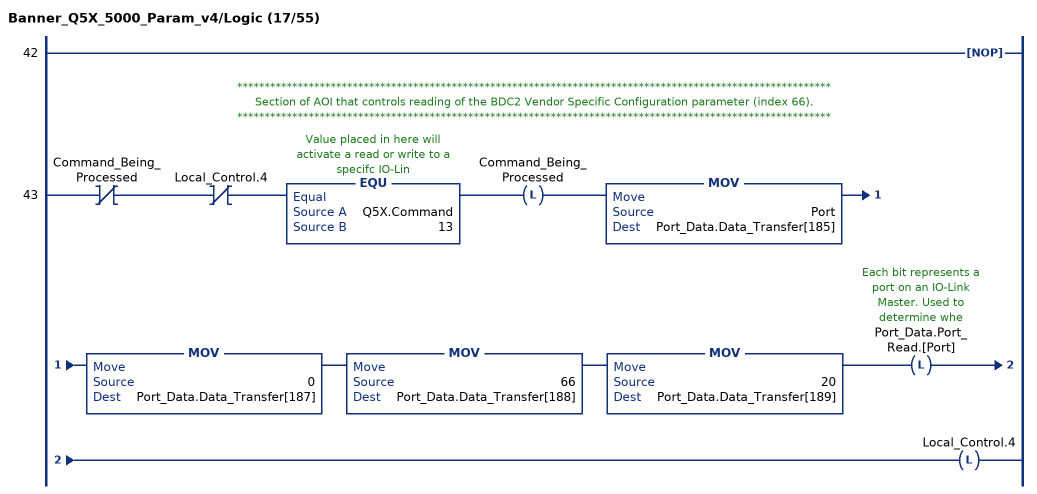
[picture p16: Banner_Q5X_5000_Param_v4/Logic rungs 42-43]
   42: NOP();
   // ************************************************************************************************************
   // Section of AOI that controls reading of the BDC2 Vendor Specific Configuration parameter (index 66).
   // ************************************************************************************************************
   43: XIO(Command_Being_Processed)XIO(Local_Control.4)EQU(Q5X.Command,13)OTL(Command_Being_Processed)MOV(Port,Port_Data.Data_Transfer[185])MOV(0,Port_Data.Data_Transfer[187])MOV(66,Port_Data.Data_Transfer[188])MOV(20,Port_Data.Data_Transfer[189])OTL(Port_Data.Port_Read.[Port])OTL(Local_Control.4);
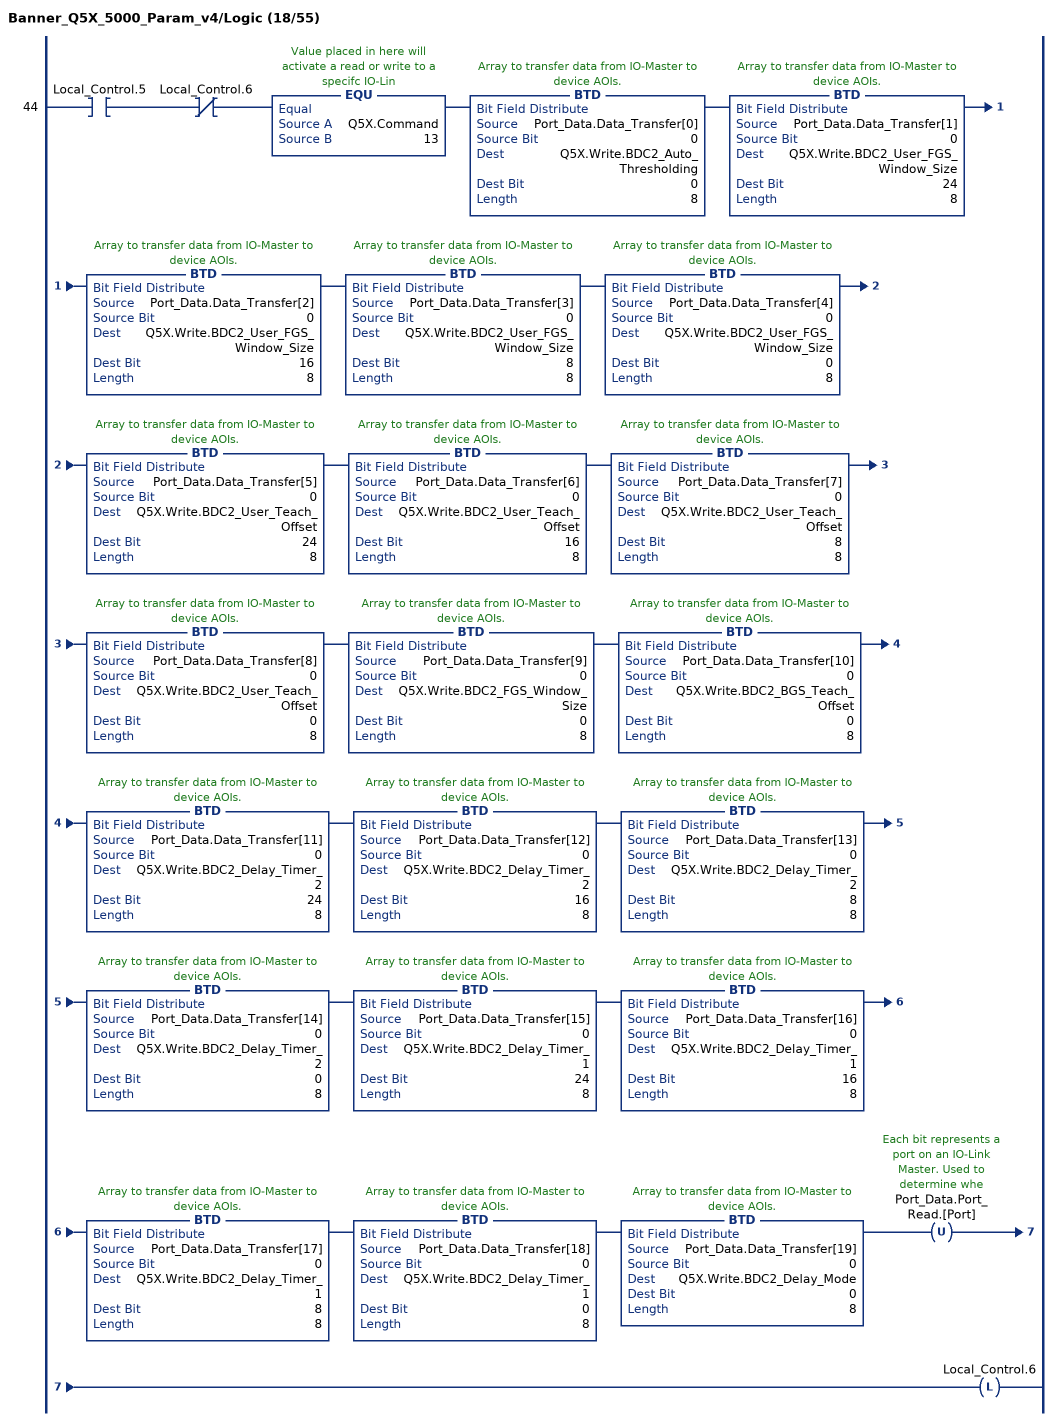
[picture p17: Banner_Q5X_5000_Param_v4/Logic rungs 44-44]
   44: XIC(Local_Control.5)XIO(Local_Control.6)EQU(Q5X.Command,13)BTD(Port_Data.Data_Transfer[0],0,Q5X.Write.BDC2_Auto_Thresholding,0,8)BTD(Port_Data.Data_Transfer[1],0,Q5X.Write.BDC2_User_FGS_Window_Size,24,8)BTD(Port_Data.Data_Transfer[2],0,Q5X.Write.BDC2_User_FGS_Window_Size,16,8)BTD(Port_Data.Data_Transfer[3],0,Q5X.Write.BDC2_User_FGS_Window_Size,8,8)BTD(Port_Data.Data_Transfer[4],0,Q5X.Write.BDC2_User_FGS_Window_Size,0,8)BTD(Port_Data.Data_Transfer[5],0,Q5X.Write.BDC2_User_Teach_Offset,24,8)BTD(Port_Data.Data_Transfer[6],0,Q5X.Write.BDC2_User_Teach_Offset,16,8)BTD(Port_Data.Data_Transfer[7],0,Q5X.Write.BDC2_User_Teach_Offset,8,8)BTD(Port_Data.Data_Transfer[8],0,Q5X.Write.BDC2_User_Teach_Offset,0,8)BTD(Port_Data.Data_Transfer[9],0,Q5X.Write.BDC2_FGS_Window_Size,0,8)BTD(Port_Data.Data_Transfer[10],0,Q5X.Write.BDC2_BGS_Teach_Offset,0,8)BTD(Port_Data.Data_Transfer[11],0,Q5X.Write.BDC2_Delay_Timer_2,24,8)BTD(Port_Data.Data_Transfer[12],0,Q5X.Write.BDC2_Delay_Timer_2,16,8)BTD(Port_Data.Data_Transfer[13],0,Q5X.Write.BDC2_Delay_Timer_2,8,8)BTD(Port_Data.Data_Transfer[14],0,Q5X.Write.BDC2_Delay_Timer_2,0,8)BTD(Port_Data.Data_Transfer[15],0,Q5X.Write.BDC2_Delay_Timer_1,24,8)BTD(Port_Data.Data_Transfer[16],0,Q5X.Write.BDC2_Delay_Timer_1,16,8)BTD(Port_Data.Data_Transfer[17],0,Q5X.Write.BDC2_Delay_Timer_1,8,8)BTD(Port_Data.Data_Transfer[18],0,Q5X.Write.BDC2_Delay_Timer_1,0,8)BTD(Port_Data.Data_Transfer[19],0,Q5X.Write.BDC2_Delay_Mode,0,8)OTU(Port_Data.Port_Read.[Port])OTL(Local_Control.6);
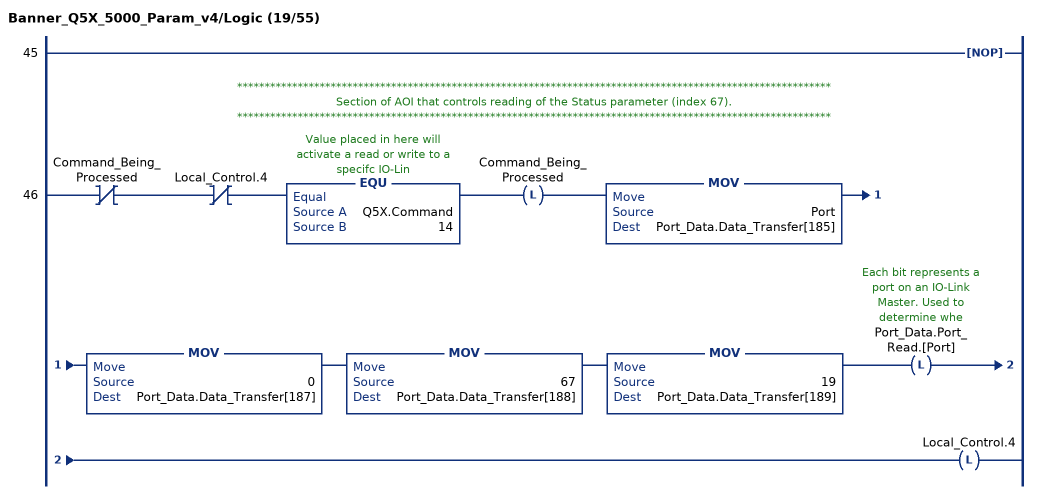
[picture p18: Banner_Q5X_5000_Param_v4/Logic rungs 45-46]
   45: NOP();
   // ************************************************************************************************************
   // Section of AOI that controls reading of the Status parameter (index 67).
   // ************************************************************************************************************
   46: XIO(Command_Being_Processed)XIO(Local_Control.4)EQU(Q5X.Command,14)OTL(Command_Being_Processed)MOV(Port,Port_Data.Data_Transfer[185])MOV(0,Port_Data.Data_Transfer[187])MOV(67,Port_Data.Data_Transfer[188])MOV(19,Port_Data.Data_Transfer[189])OTL(Port_Data.Port_Read.[Port])OTL(Local_Control.4);
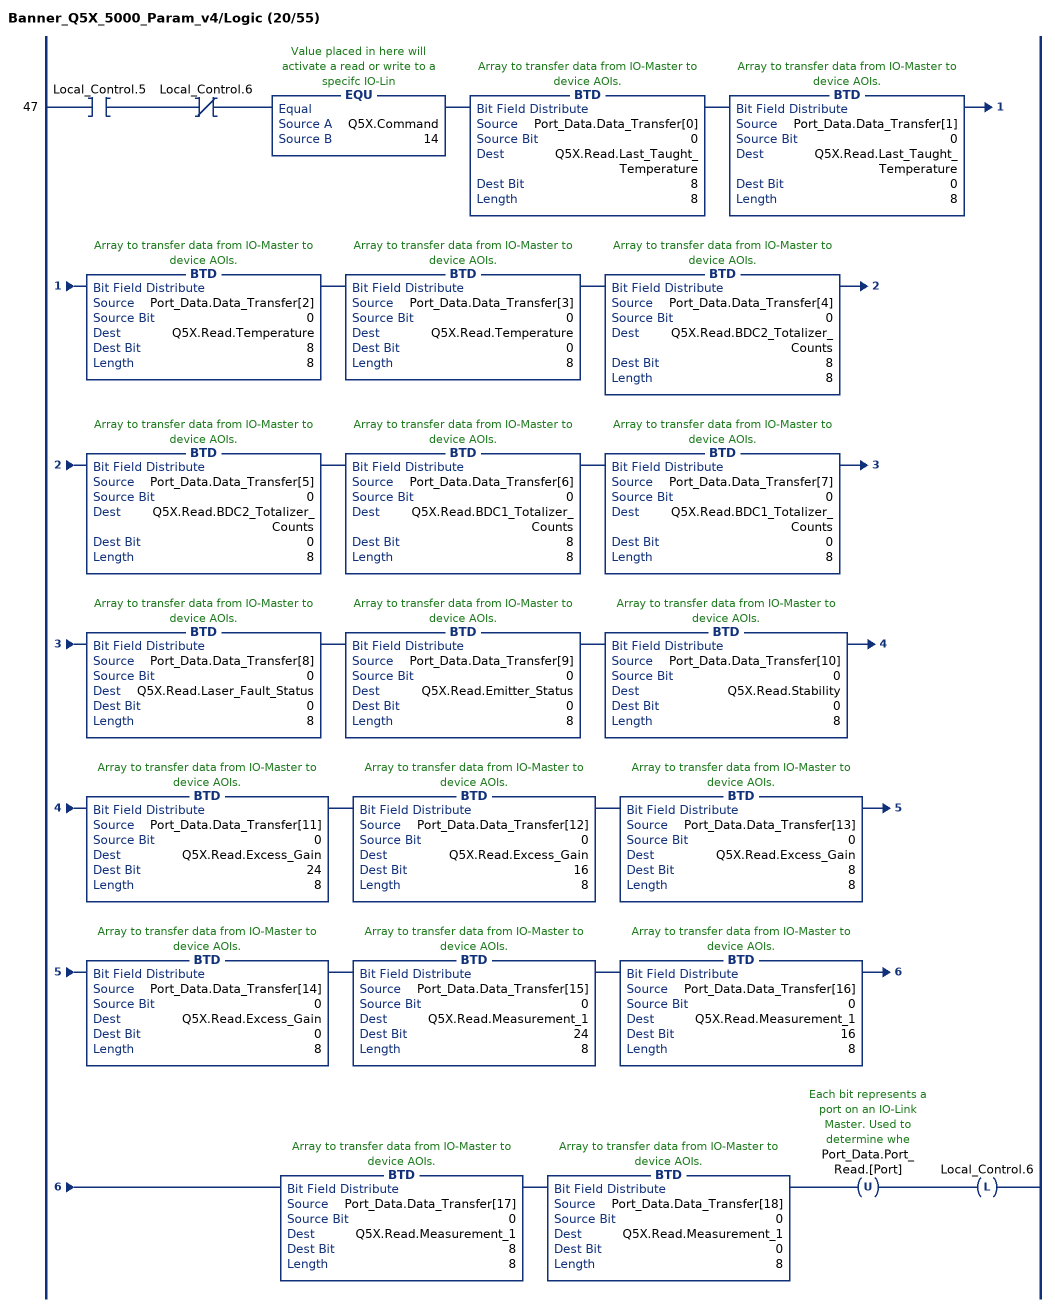
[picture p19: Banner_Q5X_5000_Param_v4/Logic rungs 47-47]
   47: XIC(Local_Control.5)XIO(Local_Control.6)EQU(Q5X.Command,14)BTD(Port_Data.Data_Transfer[0],0,Q5X.Read.Last_Taught_Temperature,8,8)BTD(Port_Data.Data_Transfer[1],0,Q5X.Read.Last_Taught_Temperature,0,8)BTD(Port_Data.Data_Transfer[2],0,Q5X.Read.Temperature,8,8)BTD(Port_Data.Data_Transfer[3],0,Q5X.Read.Temperature,0,8)BTD(Port_Data.Data_Transfer[4],0,Q5X.Read.BDC2_Totalizer_Counts,8,8)BTD(Port_Data.Data_Transfer[5],0,Q5X.Read.BDC2_Totalizer_Counts,0,8)BTD(Port_Data.Data_Transfer[6],0,Q5X.Read.BDC1_Totalizer_Counts,8,8)BTD(Port_Data.Data_Transfer[7],0,Q5X.Read.BDC1_Totalizer_Counts,0,8)BTD(Port_Data.Data_Transfer[8],0,Q5X.Read.Laser_Fault_Status,0,8)BTD(Port_Data.Data_Transfer[9],0,Q5X.Read.Emitter_Status,0,8)BTD(Port_Data.Data_Transfer[10],0,Q5X.Read.Stability,0,8)BTD(Port_Data.Data_Transfer[11],0,Q5X.Read.Excess_Gain,24,8)BTD(Port_Data.Data_Transfer[12],0,Q5X.Read.Excess_Gain,16,8)BTD(Port_Data.Data_Transfer[13],0,Q5X.Read.Excess_Gain,8,8)BTD(Port_Data.Data_Transfer[14],0,Q5X.Read.Excess_Gain,0,8)BTD(Port_Data.Data_Transfer[15],0,Q5X.Read.Measurement_1,24,8)BTD(Port_Data.Data_Transfer[16],0,Q5X.Read.Measurement_1,16,8)BTD(Port_Data.Data_Transfer[17],0,Q5X.Read.Measurement_1,8,8)BTD(Port_Data.Data_Transfer[18],0,Q5X.Read.Measurement_1,0,8)OTU(Port_Data.Port_Read.[Port])OTL(Local_Control.6);
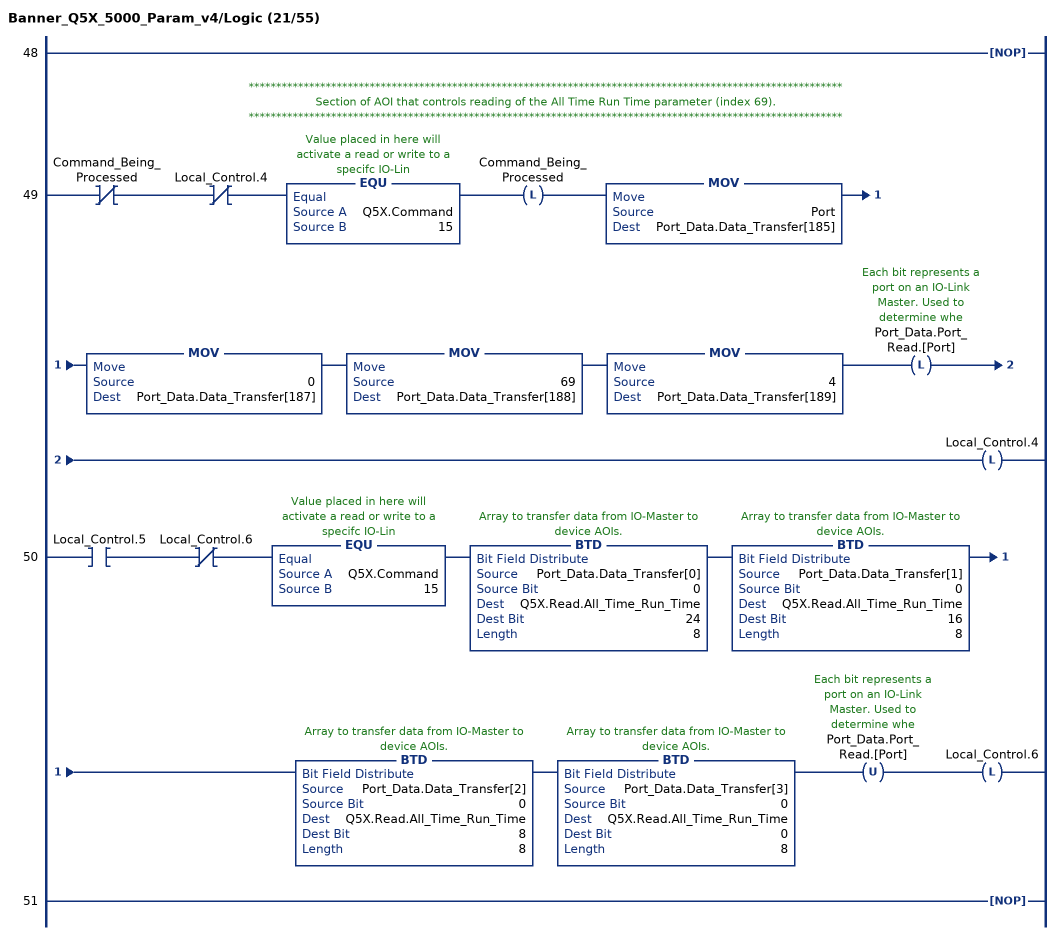
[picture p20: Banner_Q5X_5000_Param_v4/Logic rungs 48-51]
   48: NOP();
   // ************************************************************************************************************
   // Section of AOI that controls reading of the All Time Run Time parameter (index 69).
   // ************************************************************************************************************
   49: XIO(Command_Being_Processed)XIO(Local_Control.4)EQU(Q5X.Command,15)OTL(Command_Being_Processed)MOV(Port,Port_Data.Data_Transfer[185])MOV(0,Port_Data.Data_Transfer[187])MOV(69,Port_Data.Data_Transfer[188])MOV(4,Port_Data.Data_Transfer[189])OTL(Port_Data.Port_Read.[Port])OTL(Local_Control.4);
   50: XIC(Local_Control.5)XIO(Local_Control.6)EQU(Q5X.Command,15)BTD(Port_Data.Data_Transfer[0],0,Q5X.Read.All_Time_Run_Time,24,8)BTD(Port_Data.Data_Transfer[1],0,Q5X.Read.All_Time_Run_Time,16,8)BTD(Port_Data.Data_Transfer[2],0,Q5X.Read.All_Time_Run_Time,8,8)BTD(Port_Data.Data_Transfer[3],0,Q5X.Read.All_Time_Run_Time,0,8)OTU(Port_Data.Port_Read.[Port])OTL(Local_Control.6);
   51: NOP();
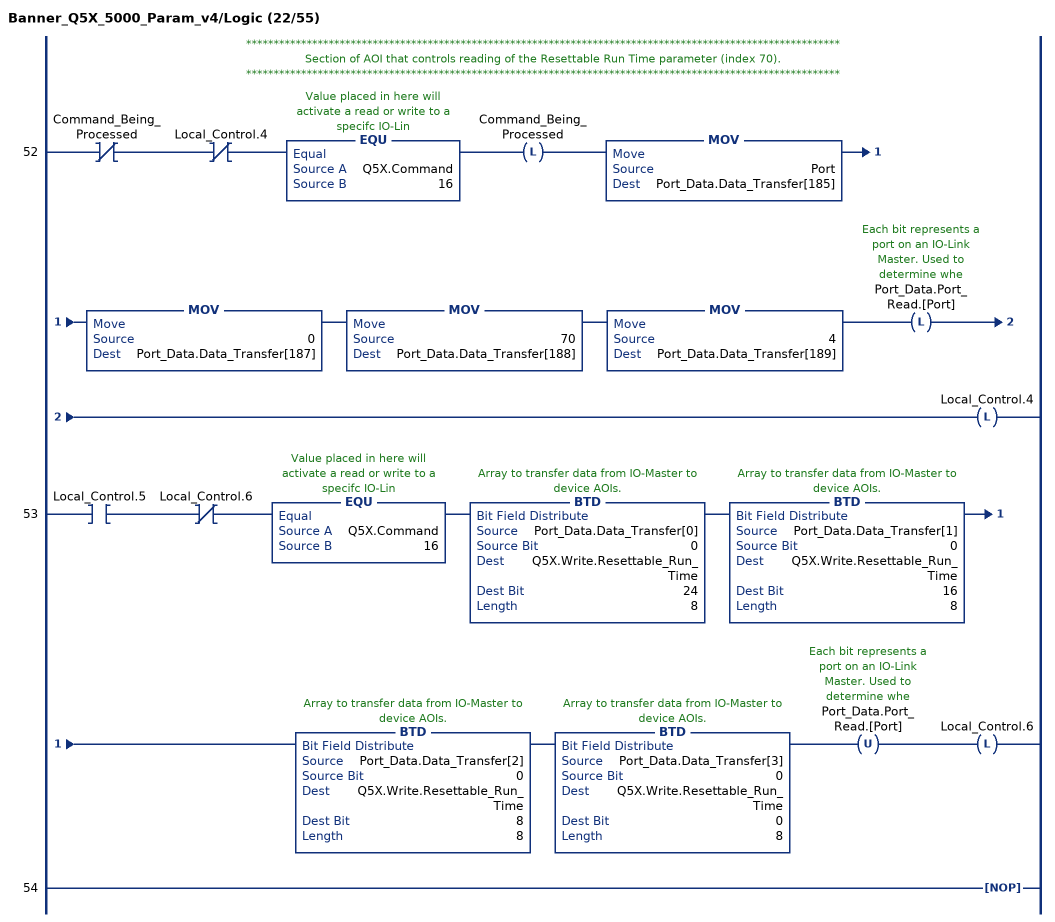
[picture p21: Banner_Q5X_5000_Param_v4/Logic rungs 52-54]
   // ************************************************************************************************************
   // Section of AOI that controls reading of the Resettable Run Time parameter (index 70).
   // ************************************************************************************************************
   52: XIO(Command_Being_Processed)XIO(Local_Control.4)EQU(Q5X.Command,16)OTL(Command_Being_Processed)MOV(Port,Port_Data.Data_Transfer[185])MOV(0,Port_Data.Data_Transfer[187])MOV(70,Port_Data.Data_Transfer[188])MOV(4,Port_Data.Data_Transfer[189])OTL(Port_Data.Port_Read.[Port])OTL(Local_Control.4);
   53: XIC(Local_Control.5)XIO(Local_Control.6)EQU(Q5X.Command,16)BTD(Port_Data.Data_Transfer[0],0,Q5X.Write.Resettable_Run_Time,24,8)BTD(Port_Data.Data_Transfer[1],0,Q5X.Write.Resettable_Run_Time,16,8)BTD(Port_Data.Data_Transfer[2],0,Q5X.Write.Resettable_Run_Time,8,8)BTD(Port_Data.Data_Transfer[3],0,Q5X.Write.Resettable_Run_Time,0,8)OTU(Port_Data.Port_Read.[Port])OTL(Local_Control.6);
   54: NOP();
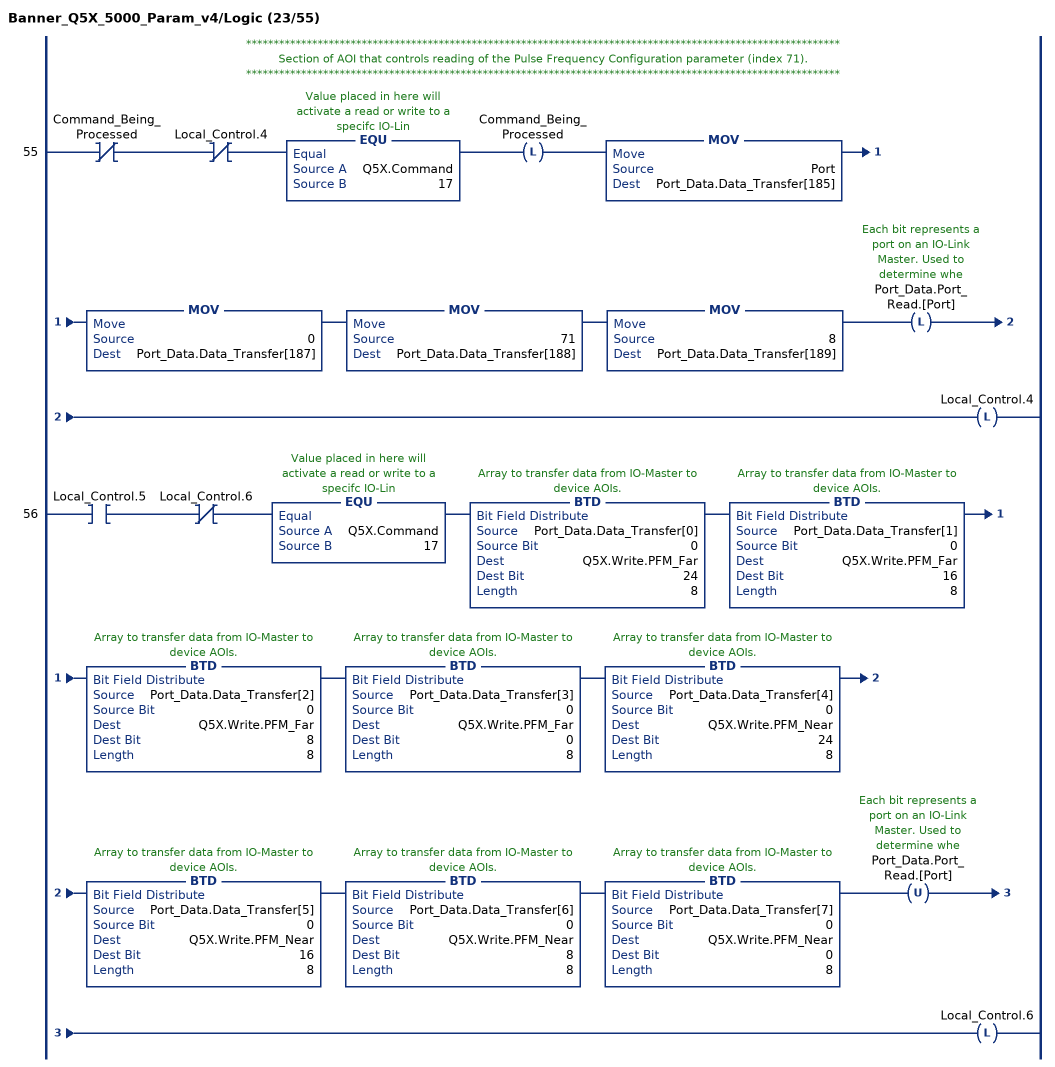
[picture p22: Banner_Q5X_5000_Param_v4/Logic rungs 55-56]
   // ************************************************************************************************************
   // Section of AOI that controls reading of the Pulse Frequency Configuration parameter (index 71).
   // ************************************************************************************************************
   55: XIO(Command_Being_Processed)XIO(Local_Control.4)EQU(Q5X.Command,17)OTL(Command_Being_Processed)MOV(Port,Port_Data.Data_Transfer[185])MOV(0,Port_Data.Data_Transfer[187])MOV(71,Port_Data.Data_Transfer[188])MOV(8,Port_Data.Data_Transfer[189])OTL(Port_Data.Port_Read.[Port])OTL(Local_Control.4);
   56: XIC(Local_Control.5)XIO(Local_Control.6)EQU(Q5X.Command,17)BTD(Port_Data.Data_Transfer[0],0,Q5X.Write.PFM_Far,24,8)BTD(Port_Data.Data_Transfer[1],0,Q5X.Write.PFM_Far,16,8)BTD(Port_Data.Data_Transfer[2],0,Q5X.Write.PFM_Far,8,8)BTD(Port_Data.Data_Transfer[3],0,Q5X.Write.PFM_Far,0,8)BTD(Port_Data.Data_Transfer[4],0,Q5X.Write.PFM_Near,24,8)BTD(Port_Data.Data_Transfer[5],0,Q5X.Write.PFM_Near,16,8)BTD(Port_Data.Data_Transfer[6],0,Q5X.Write.PFM_Near,8,8)BTD(Port_Data.Data_Transfer[7],0,Q5X.Write.PFM_Near,0,8)OTU(Port_Data.Port_Read.[Port])OTL(Local_Control.6);
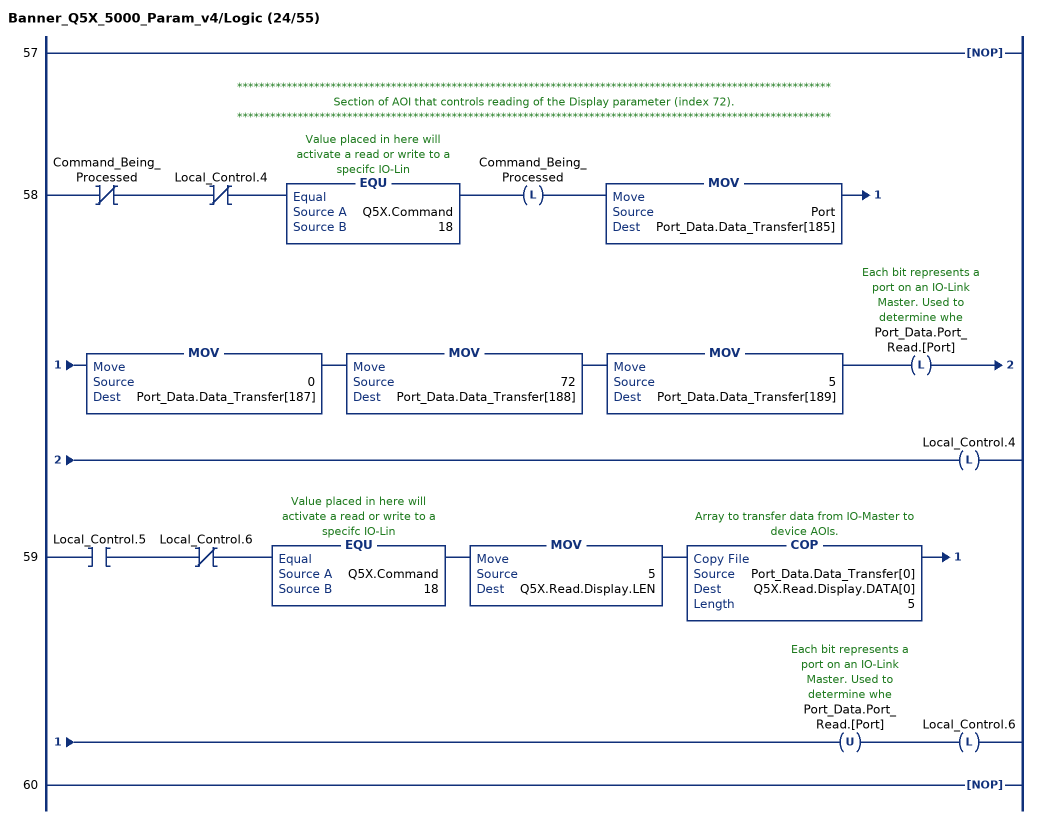
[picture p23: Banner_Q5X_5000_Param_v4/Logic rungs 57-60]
   57: NOP();
   // ************************************************************************************************************
   // Section of AOI that controls reading of the Display parameter (index 72).
   // ************************************************************************************************************
   58: XIO(Command_Being_Processed)XIO(Local_Control.4)EQU(Q5X.Command,18)OTL(Command_Being_Processed)MOV(Port,Port_Data.Data_Transfer[185])MOV(0,Port_Data.Data_Transfer[187])MOV(72,Port_Data.Data_Transfer[188])MOV(5,Port_Data.Data_Transfer[189])OTL(Port_Data.Port_Read.[Port])OTL(Local_Control.4);
   59: XIC(Local_Control.5)XIO(Local_Control.6)EQU(Q5X.Command,18)MOV(5,Q5X.Read.Display.LEN)COP(Port_Data.Data_Transfer[0],Q5X.Read.Display.DATA[0],5)OTU(Port_Data.Port_Read.[Port])OTL(Local_Control.6);
   60: NOP();
